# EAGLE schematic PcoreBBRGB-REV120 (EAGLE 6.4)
Assembly variants: FERT1S, FERT1B

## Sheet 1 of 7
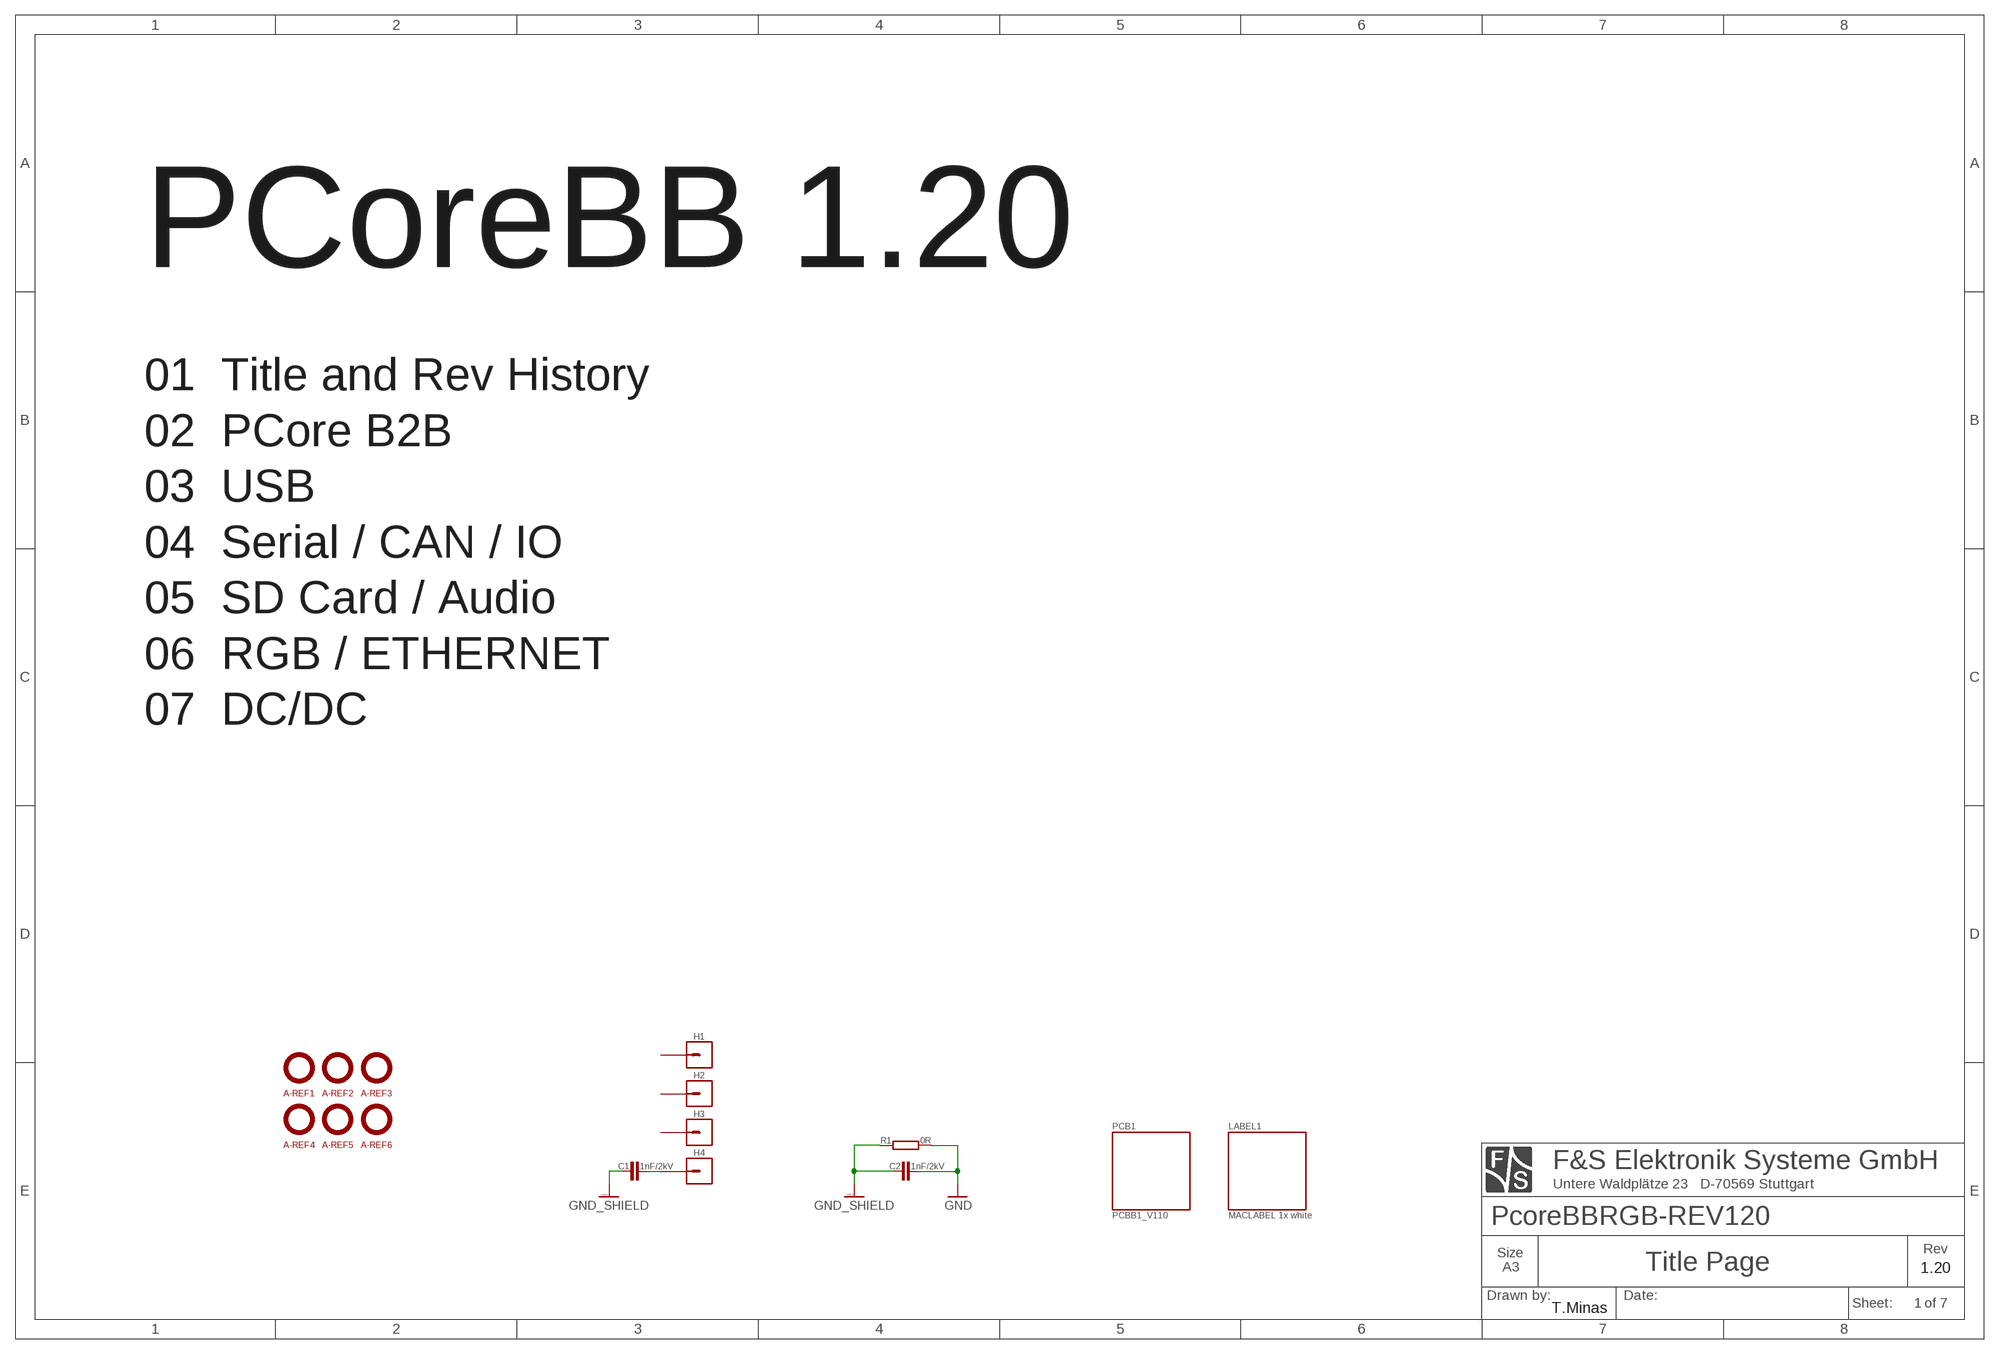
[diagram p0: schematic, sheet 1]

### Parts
A-REF1  A-REF  [A-REF]
A-REF2  A-REF  [A-REF]
A-REF3  A-REF  [A-REF]
A-REF4  A-REF  [A-REF]
A-REF5  A-REF  [A-REF]
A-REF6  A-REF  [A-REF]
C1  1nF/2kV  C1206-H  [1206]  (not fitted in variant FERT1B)
C2  1nF/2kV  C1206-H  [1206]  (not fitted in variant FERT1B)
H1  HOLE-3.2X6  [HOLE-3.2X6]  (not fitted in variant FERT1B)
H2  HOLE-3.2X6  [HOLE-3.2X6]  (not fitted in variant FERT1B)
H3  HOLE-3.2X6  [HOLE-3.2X6]  (not fitted in variant FERT1B)
H4  HOLE-3.2X6  [HOLE-3.2X6]  (not fitted in variant FERT1B)
R1  0R  R0805-H  [0805]  (not fitted in variant FERT1B)

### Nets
GND: C2.2 R1.2 ; also sheet 2,3,4,5,6,7
GND_SHIELD: C1.1 C2.1 R1.1 ; also sheet 3,6
N$1: C1.2 H4.P$1
Unconnected: H1.P$1 H2.P$1 H3.P$1

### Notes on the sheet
- PCoreBB 1.20
- 01  Title and Rev History
  02  PCore B2B
  03  USB
  04  Serial / CAN / IO
  05  SD Card / Audio
  06  RGB / ETHERNET
  07  DC/DC
- 1.20
- T.Minas

## Sheet 2 of 7: PicoCORE
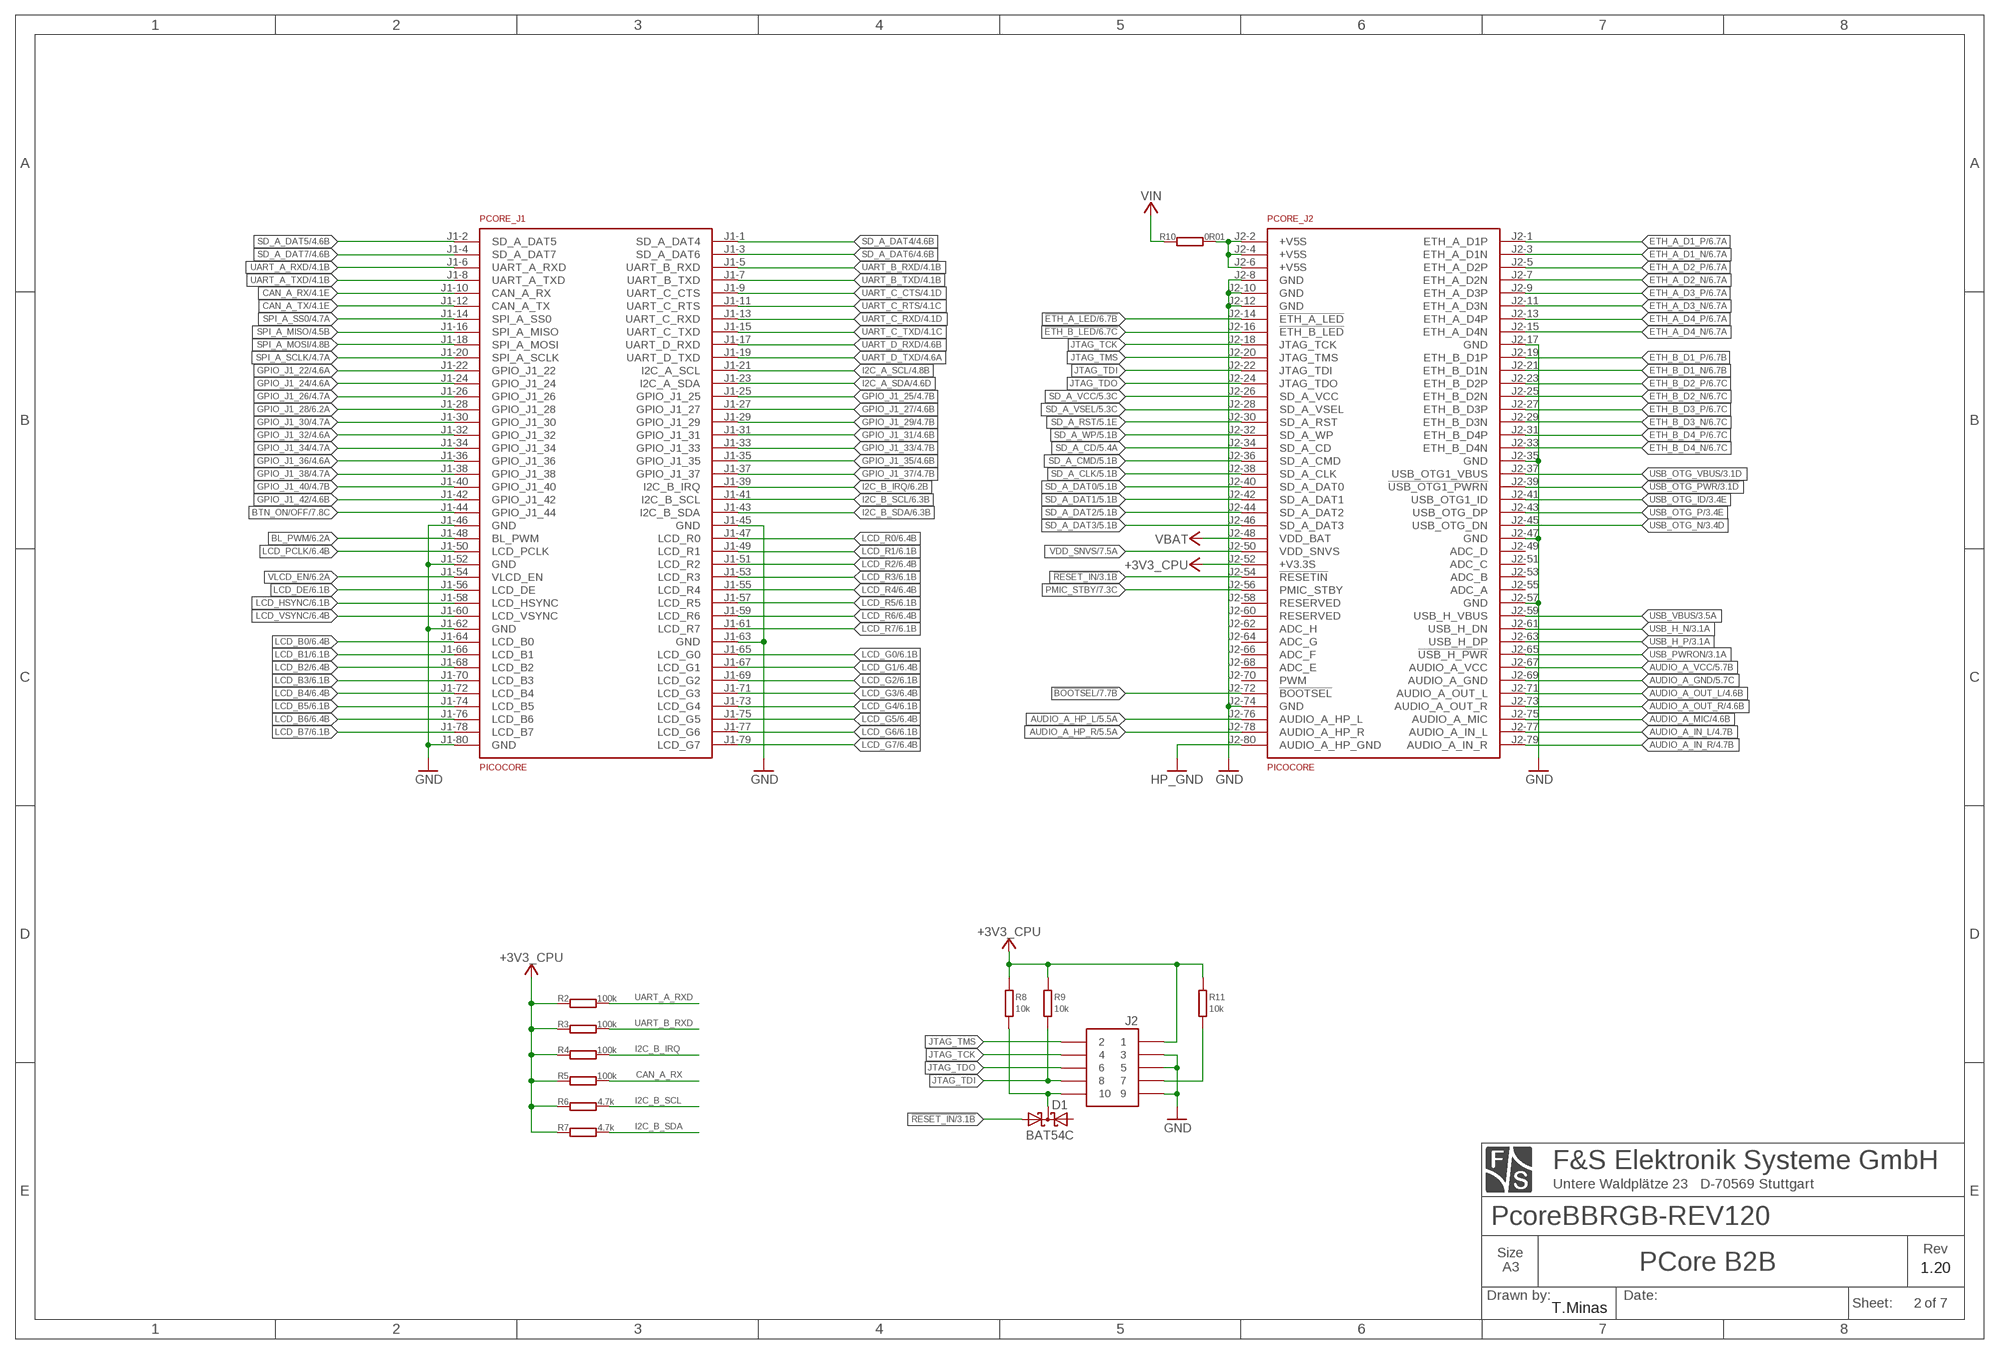
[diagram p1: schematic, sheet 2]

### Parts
D1  BAT54C  [SOT23]  (not fitted in variant FERT1B)
J2  CON-10-POL.-SMD-127  [10-POL.SMD-127]  (not fitted in variant FERT1B)
PCORE_  PICOCORE  [PICOCORE]  (not fitted in variant FERT1B)
R2  100k  R0402  [0402]  (not fitted in variant FERT1B)
R3  100k  R0402  [0402]  (not fitted in variant FERT1B)
R4  100k  R0402  [0402]  (not fitted in variant FERT1B)
R5  100k  R0402  [0402]  (not fitted in variant FERT1B)
R6  4.7k  R0402  [0402]  (not fitted in variant FERT1B)
R7  4.7k  R0402  [0402]  (not fitted in variant FERT1B)
R8  10k  R0402-V  [0402@1]  (not fitted in variant FERT1B)
R9  10k  R0402-V  [0402@1]  (not fitted in variant FERT1B)
R10  0R01  R0805-H  [0805]  (not fitted in variant FERT1B)
R11  10k  R0402-V  [0402@1]  (not fitted in variant FERT1B)

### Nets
!BOOTSEL: PCORE_.J2-72(J2:!BOOTSEL) ; also sheet 7
!ETH_A_LED: PCORE_.J2-14(J2:!ETH_A_LED) ; also sheet 6
!ETH_B_LED: PCORE_.J2-16(J2:!ETH_B_LED) ; also sheet 6
!JTAG_SRST: D1.3(CC) J2.10 R8.1
!RESET_IN: D1.1(A1) PCORE_.J2-54(J2:!RESETIN) ; also sheet 3,7
!USB_OTG_PWR: PCORE_.J2-39(J2:!USB_OTG1_PWRN) ; also sheet 3
+3V3_CPU [+3V3]: J2.1 PCORE_.J2-52(J2:+V3.3S) R2.1 R3.1 R4.1 R5.1 R6.1 R7.1 R8.2 R9.2 R11.2 ; also sheet 3,6,7
AUDIO_A_GND: PCORE_.J2-69(J2:AUDIO_A_GND) ; also sheet 5
AUDIO_A_HP_L: PCORE_.J2-76(J2:AUDIO_A_HP_L) ; also sheet 5
AUDIO_A_HP_R: PCORE_.J2-78(J2:AUDIO_A_HP_R) ; also sheet 5
AUDIO_A_IN_L: PCORE_.J2-77(J2:AUDIO_A_IN_L) ; also sheet 4
AUDIO_A_IN_R: PCORE_.J2-79(J2:AUDIO_A_IN_R) ; also sheet 4
AUDIO_A_MIC: PCORE_.J2-75(J2:AUDIO_A_MIC) ; also sheet 4,5
AUDIO_A_OUT_L: PCORE_.J2-71(J2:AUDIO_A_OUT_L) ; also sheet 4
AUDIO_A_OUT_R: PCORE_.J2-73(J2:AUDIO_A_OUT_R) ; also sheet 4
AUDIO_A_VCC: PCORE_.J2-67(J2:AUDIO_A_VCC) ; also sheet 5
BL_PWM: PCORE_.J1-48(J1:BL_PWM) ; also sheet 6
BTN_ON/OFF: PCORE_.J1-44(J1:GPIO_J1_44) ; also sheet 7
CAN_A_RX: PCORE_.J1-10(J1:CAN_A_RX) R5.2 ; also sheet 4
CAN_A_TX: PCORE_.J1-12(J1:CAN_A_TX) ; also sheet 4
ETH_A_D1_N [ETHERNET]: PCORE_.J2-3(J2:ETH_A_D1N) ; also sheet 6
ETH_A_D1_P [ETHERNET]: PCORE_.J2-1(J2:ETH_A_D1P) ; also sheet 6
ETH_A_D2_N [ETHERNET]: PCORE_.J2-7(J2:ETH_A_D2N) ; also sheet 6
ETH_A_D2_P [ETHERNET]: PCORE_.J2-5(J2:ETH_A_D2P) ; also sheet 6
ETH_A_D3_N [ETHERNET]: PCORE_.J2-11(J2:ETH_A_D3N) ; also sheet 6
ETH_A_D3_P [ETHERNET]: PCORE_.J2-9(J2:ETH_A_D3P) ; also sheet 6
ETH_A_D4_N [ETHERNET]: PCORE_.J2-15(J2:ETH_A_D4N) ; also sheet 6
ETH_A_D4_P [ETHERNET]: PCORE_.J2-13(J2:ETH_A_D4P) ; also sheet 6
ETH_B_D1_N [ETHERNET]: PCORE_.J2-21(J2:ETH_B_D1N) ; also sheet 6
ETH_B_D1_P [ETHERNET]: PCORE_.J2-19(J2:ETH_B_D1P) ; also sheet 6
ETH_B_D2_N [ETHERNET]: PCORE_.J2-25(J2:ETH_B_D2N) ; also sheet 6
ETH_B_D2_P [ETHERNET]: PCORE_.J2-23(J2:ETH_B_D2P) ; also sheet 6
ETH_B_D3_N [ETHERNET]: PCORE_.J2-29(J2:ETH_B_D3N) ; also sheet 6
ETH_B_D3_P [ETHERNET]: PCORE_.J2-27(J2:ETH_B_D3P) ; also sheet 6
ETH_B_D4_N [ETHERNET]: PCORE_.J2-33(J2:ETH_B_D4N) ; also sheet 6
ETH_B_D4_P [ETHERNET]: PCORE_.J2-31(J2:ETH_B_D4P) ; also sheet 6
GND: J2.3 J2.5 J2.9 PCORE_.J1-45(J1:GND) PCORE_.J1-46(J1:GND) PCORE_.J1-52(J1:GND) PCORE_.J1-62(J1:GND) PCORE_.J1-63(J1:GND) PCORE_.J1-80(J1:GND) PCORE_.J2-8(J2:GND) PCORE_.J2-10(J2:GND) PCORE_.J2-12(J2:GND) PCORE_.J2-17(J2:GND) PCORE_.J2-35(J2:GND) PCORE_.J2-47(J2:GND) PCORE_.J2-57(J2:GND) PCORE_.J2-74(J2:GND) ; also sheet 1,3,4,5,6,7
GPIO_J1_22: PCORE_.J1-22(J1:GPIO_J1_22) ; also sheet 4
GPIO_J1_24: PCORE_.J1-24(J1:GPIO_J1_24) ; also sheet 4
GPIO_J1_25: PCORE_.J1-25(J1:GPIO_J1_25) ; also sheet 4
GPIO_J1_26: PCORE_.J1-26(J1:GPIO_J1_26) ; also sheet 4
GPIO_J1_27: PCORE_.J1-27(J1:GPIO_J1_27) ; also sheet 4
GPIO_J1_28: PCORE_.J1-28(J1:GPIO_J1_28) ; also sheet 6
GPIO_J1_29: PCORE_.J1-29(J1:GPIO_J1_29) ; also sheet 4
GPIO_J1_30: PCORE_.J1-30(J1:GPIO_J1_30) ; also sheet 4
GPIO_J1_31: PCORE_.J1-31(J1:GPIO_J1_31) ; also sheet 4
GPIO_J1_32: PCORE_.J1-32(J1:GPIO_J1_32) ; also sheet 4
GPIO_J1_33: PCORE_.J1-33(J1:GPIO_J1_33) ; also sheet 4
GPIO_J1_34: PCORE_.J1-34(J1:GPIO_J1_34) ; also sheet 4
GPIO_J1_35: PCORE_.J1-35(J1:GPIO_J1_35) ; also sheet 4
GPIO_J1_36: PCORE_.J1-36(J1:GPIO_J1_36) ; also sheet 4
GPIO_J1_37: PCORE_.J1-37(J1:GPIO_J1_37) ; also sheet 4
GPIO_J1_38: PCORE_.J1-38(J1:GPIO_J1_38) ; also sheet 4
GPIO_J1_40: PCORE_.J1-40(J1:GPIO_J1_40) ; also sheet 4
GPIO_J1_42: PCORE_.J1-42(J1:GPIO_J1_42) ; also sheet 4
HP_GND: PCORE_.J2-80(J2:AUDIO_A_HP_GND) ; also sheet 5
I2C_A_SCL: PCORE_.J1-21(J1:I2C_A_SCL) ; also sheet 4
I2C_A_SDA: PCORE_.J1-23(J1:I2C_A_SDA) ; also sheet 4
I2C_B_IRQ: PCORE_.J1-39(J1:I2C_B_IRQ) R4.2 ; also sheet 6
I2C_B_SCL: PCORE_.J1-41(J1:I2C_B_SCL) R6.2 ; also sheet 6
I2C_B_SDA: PCORE_.J1-43(J1:I2C_B_SDA) R7.2 ; also sheet 6
JTAG_TCK: J2.4 PCORE_.J2-18(J2:JTAG_TCK)
JTAG_TDI: J2.8 PCORE_.J2-22(J2:JTAG_TDI) R9.1
JTAG_TDO: J2.6 PCORE_.J2-24(J2:JTAG_TDO)
JTAG_TMS: J2.2 PCORE_.J2-20(J2:JTAG_TMS)
LCD_B0: PCORE_.J1-64(J1:LCD_B0) ; also sheet 6
LCD_B1: PCORE_.J1-66(J1:LCD_B1) ; also sheet 6
LCD_B2: PCORE_.J1-68(J1:LCD_B2) ; also sheet 6
LCD_B3: PCORE_.J1-70(J1:LCD_B3) ; also sheet 6
LCD_B4: PCORE_.J1-72(J1:LCD_B4) ; also sheet 6
LCD_B5: PCORE_.J1-74(J1:LCD_B5) ; also sheet 6
LCD_B6: PCORE_.J1-76(J1:LCD_B6) ; also sheet 6
LCD_B7: PCORE_.J1-78(J1:LCD_B7) ; also sheet 6
LCD_DE: PCORE_.J1-56(J1:LCD_DE) ; also sheet 6
LCD_G0: PCORE_.J1-65(J1:LCD_G0) ; also sheet 6
LCD_G1: PCORE_.J1-67(J1:LCD_G1) ; also sheet 6
LCD_G2: PCORE_.J1-69(J1:LCD_G2) ; also sheet 6
LCD_G3: PCORE_.J1-71(J1:LCD_G3) ; also sheet 6
LCD_G4: PCORE_.J1-73(J1:LCD_G4) ; also sheet 6
LCD_G5: PCORE_.J1-75(J1:LCD_G5) ; also sheet 6
LCD_G6: PCORE_.J1-77(J1:LCD_G6) ; also sheet 6
LCD_G7: PCORE_.J1-79(J1:LCD_G7) ; also sheet 6
LCD_HSYNC: PCORE_.J1-58(J1:LCD_HSYNC) ; also sheet 6
LCD_PCLK: PCORE_.J1-50(J1:LCD_PCLK) ; also sheet 6
LCD_R0: PCORE_.J1-47(J1:LCD_R0) ; also sheet 6
LCD_R1: PCORE_.J1-49(J1:LCD_R1) ; also sheet 6
LCD_R2: PCORE_.J1-51(J1:LCD_R2) ; also sheet 6
LCD_R3: PCORE_.J1-53(J1:LCD_R3) ; also sheet 6
LCD_R4: PCORE_.J1-55(J1:LCD_R4) ; also sheet 6
LCD_R5: PCORE_.J1-57(J1:LCD_R5) ; also sheet 6
LCD_R6: PCORE_.J1-59(J1:LCD_R6) ; also sheet 6
LCD_R7: PCORE_.J1-61(J1:LCD_R7) ; also sheet 6
LCD_VSYNC: PCORE_.J1-60(J1:LCD_VSYNC) ; also sheet 6
N$23: PCORE_.J2-2(J2:+V5S) PCORE_.J2-4(J2:+V5S) PCORE_.J2-6(J2:+V5S) R10.2
N$34: J2.7 R11.1
PMIC_STBY: PCORE_.J2-56(J2:PMIC_STBY) ; also sheet 7
SD_A_CD: PCORE_.J2-34(J2:SD_A_CD) ; also sheet 5
SD_A_CLK: PCORE_.J2-38(J2:SD_A_CLK) ; also sheet 5
SD_A_CMD: PCORE_.J2-36(J2:SD_A_CMD) ; also sheet 5
SD_A_DAT0: PCORE_.J2-40(J2:SD_A_DAT0) ; also sheet 5
SD_A_DAT1: PCORE_.J2-42(J2:SD_A_DAT1) ; also sheet 5
SD_A_DAT2: PCORE_.J2-44(J2:SD_A_DAT2) ; also sheet 5
SD_A_DAT3: PCORE_.J2-46(J2:SD_A_DAT3) ; also sheet 5
SD_A_DAT4: PCORE_.J1-1(J1:SD_A_DAT4) ; also sheet 4
SD_A_DAT5: PCORE_.J1-2(J1:SD_A_DAT5) ; also sheet 4
SD_A_DAT6: PCORE_.J1-3(J1:SD_A_DAT6) ; also sheet 4
SD_A_DAT7: PCORE_.J1-4(J1:SD_A_DAT7) ; also sheet 4
SD_A_RST: PCORE_.J2-30(J2:SD_A_RST) ; also sheet 5
SD_A_VCC: PCORE_.J2-26(J2:SD_A_VCC) ; also sheet 5
SD_A_VSEL: PCORE_.J2-28(J2:SD_A_VSEL) ; also sheet 5
SD_A_WP: PCORE_.J2-32(J2:SD_A_WP) ; also sheet 5
SPI_A_MISO: PCORE_.J1-16(J1:SPI_A_MISO) ; also sheet 4
SPI_A_MOSI: PCORE_.J1-18(J1:SPI_A_MOSI) ; also sheet 4
SPI_A_SCLK: PCORE_.J1-20(J1:SPI_A_SCLK) ; also sheet 4
SPI_A_SS0: PCORE_.J1-14(J1:SPI_A_SS0) ; also sheet 4
UART_A_RXD: PCORE_.J1-6(J1:UART_A_RXD) R2.2 ; also sheet 4
UART_A_TXD: PCORE_.J1-8(J1:UART_A_TXD) ; also sheet 4
UART_B_RXD: PCORE_.J1-5(J1:UART_B_RXD) R3.2 ; also sheet 4
UART_B_TXD: PCORE_.J1-7(J1:UART_B_TXD) ; also sheet 4
UART_C_CTS: PCORE_.J1-9(J1:UART_C_CTS) ; also sheet 4
UART_C_RTS: PCORE_.J1-11(J1:UART_C_RTS) ; also sheet 4
UART_C_RXD: PCORE_.J1-13(J1:UART_C_RXD) ; also sheet 4
UART_C_TXD: PCORE_.J1-15(J1:UART_C_TXD) ; also sheet 4
UART_D_RXD: PCORE_.J1-17(J1:UART_D_RXD) ; also sheet 4
UART_D_TXD: PCORE_.J1-19(J1:UART_D_TXD) ; also sheet 4
USB_H_N [USB]: PCORE_.J2-61(J2:USB_H_DN) ; also sheet 3
USB_H_P [USB]: PCORE_.J2-63(J2:USB_H_DP) ; also sheet 3
USB_OTG_ID: PCORE_.J2-41(J2:USB_OTG1_ID) ; also sheet 3
USB_OTG_N [USB]: PCORE_.J2-45(J2:USB_OTG_DN) ; also sheet 3
USB_OTG_P [USB]: PCORE_.J2-43(J2:USB_OTG_DP) ; also sheet 3
USB_OTG_VBUS: PCORE_.J2-37(J2:USB_OTG1_VBUS) ; also sheet 3
USB_PWRON: PCORE_.J2-65(J2:!USB_H_PWR) ; also sheet 3
USB_VBUS: PCORE_.J2-59(J2:USB_H_VBUS) ; also sheet 3
VBAT: PCORE_.J2-48(J2:VDD_BAT) ; also sheet 7
VDD_SNVS: PCORE_.J2-50(J2:VDD_SNVS) ; also sheet 7
VIN: R10.1 ; also sheet 5,7
VLCD_EN: PCORE_.J1-54(J1:VLCD_EN) ; also sheet 6
Unconnected: D1.2(A2) PCORE_.J2-49(J2:ADC_D) PCORE_.J2-51(J2:ADC_C) PCORE_.J2-53(J2:ADC_B) PCORE_.J2-55(J2:ADC_A) PCORE_.J2-58(J2:RESERVED) PCORE_.J2-60(J2:RESERVED) PCORE_.J2-62(J2:ADC_H) PCORE_.J2-64(J2:ADC_G) PCORE_.J2-66(J2:ADC_F) PCORE_.J2-68(J2:ADC_E) PCORE_.J2-70(J2:PWM)

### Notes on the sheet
- 1.20
- T.Minas

## Sheet 3 of 7: USB
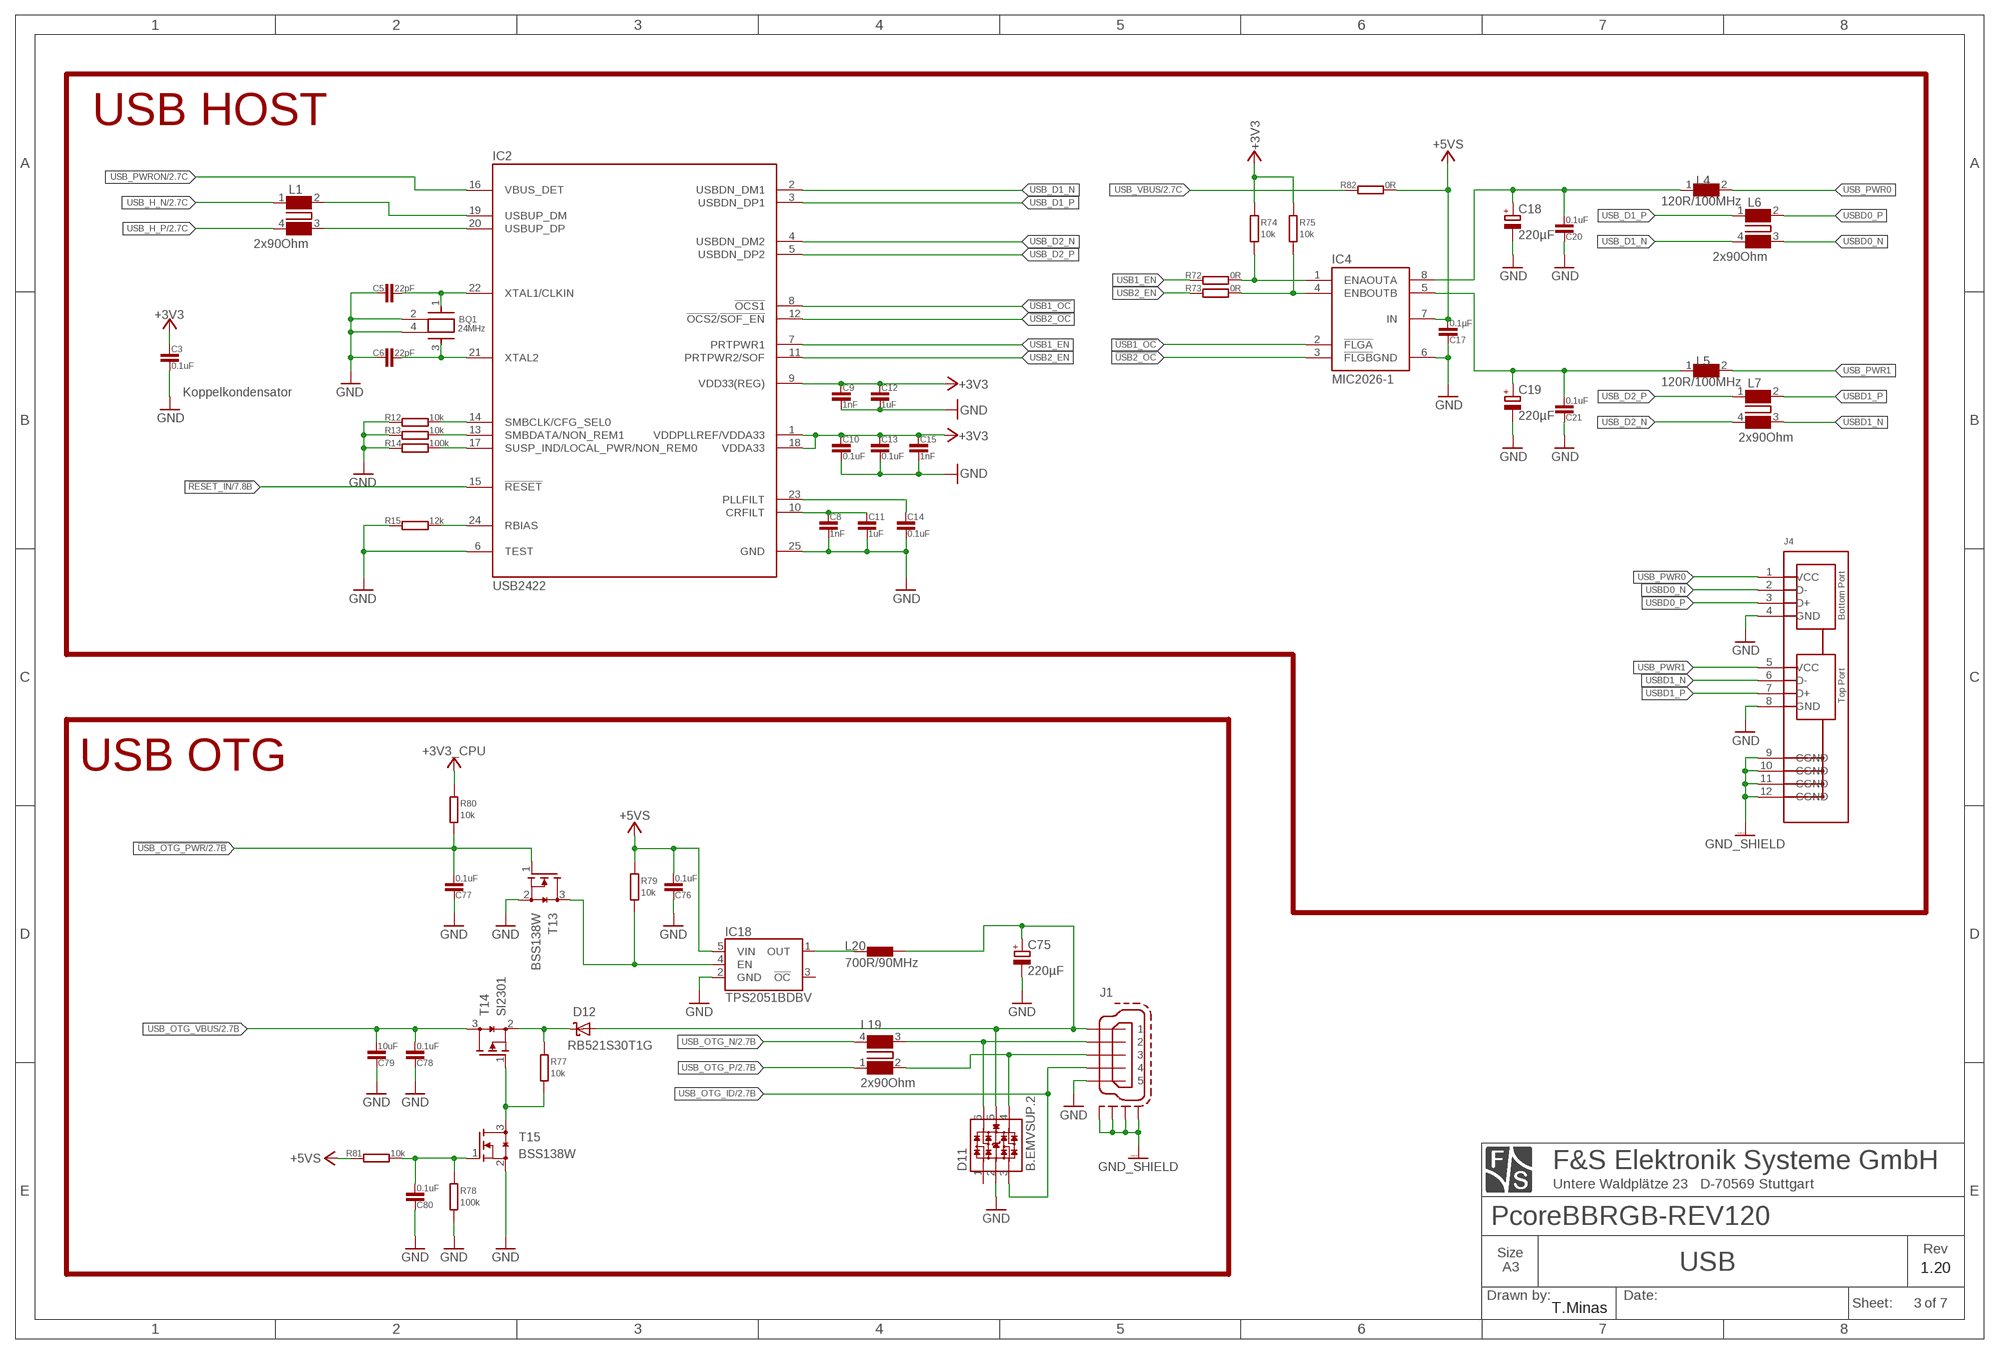
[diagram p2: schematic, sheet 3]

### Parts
BQ1  24MHz  Q-FA-238  [FA-238]  (not fitted in variant FERT1B)
C3  0.1uF  C0402-V  [0402@1]  (not fitted in variant FERT1B)
C5  22pF  C0402  [0402@1]  (not fitted in variant FERT1B)
C6  22pF  C0402  [0402@1]  (not fitted in variant FERT1B)
C8  1nF  C0402-V  [0402@1]  (not fitted in variant FERT1B)
C9  1nF  C0402-V  [0402@1]  (not fitted in variant FERT1B)
C10  0.1uF  C0402-V  [0402@1]  (not fitted in variant FERT1B)
C11  1uF  C0402-V  [0402@1]  (not fitted in variant FERT1B)
C12  1uF  C0402-V  [0402@1]  (not fitted in variant FERT1B)
C13  0.1uF  C0402-V  [0402@1]  (not fitted in variant FERT1B)
C14  0.1uF  C0402-V  [0402@1]  (not fitted in variant FERT1B)
C15  1nF  C0402-V  [0402@1]  (not fitted in variant FERT1B)
C17  0.1µF  C0402-V  [0402@1]  (not fitted in variant FERT1B)
C18  220µF  CPOL-EUSMCD  [SMC_D]  (not fitted in variant FERT1B)
C19  220µF  CPOL-EUSMCD  [SMC_D]  (not fitted in variant FERT1B)
C20  0.1uF  C0402-V  [0402@1]  (not fitted in variant FERT1B)
C21  0.1uF  C0402-V  [0402@1]  (not fitted in variant FERT1B)
C75  220µF  CPOL-EUSMCD  [SMC_D]  (not fitted in variant FERT1B)
C76  0.1uF  C0402-V  [0402@1]  (not fitted in variant FERT1B)
C77  0.1uF  C0402-V  [0402@1]  (not fitted in variant FERT1B)
C78  0.1uF  C0402-V  [0402@1]
C79  10uF  C0402-V  [0402@1]
C80  0.1uF  C0402-V  [0402@1]
D11  B.EMVSUP.2  ESD-PROTECTION-DIODE(4CHANNEL)  [SOT26]  (not fitted in variant FERT1B)
D12  RB521S30T1G  RB521S30  [SOD-523]
IC2  USB2422  [SQFN-24]  (not fitted in variant FERT1B)
IC4  MIC2026-1  MIC2026  [SO-8$1]  (not fitted in variant FERT1B)
IC18  TPS2051BDBV  [SOT23-5@1]  (not fitted in variant FERT1B)
J1  CON-MINI-USB-SCHIELD32005-201  [32005-201]  (not fitted in variant FERT1B)
J4  CON-USB-DOUBLE  [LUMBERG-2410-03]  (not fitted in variant FERT1S)
L1  2x90Ohm  WE-CNSW_HF_0805  [WE-CNSW_0805]  (not fitted in variant FERT1B)
L4  120R/100MHz  WE-CBF_HF_0402  [0402]  (not fitted in variant FERT1B)
L5  120R/100MHz  WE-CBF_HF_0402  [0402]  (not fitted in variant FERT1B)
L6  2x90Ohm  WE-CNSW_HF_0805  [WE-CNSW_0805]  (not fitted in variant FERT1B)
L7  2x90Ohm  WE-CNSW_HF_0805  [WE-CNSW_0805]  (not fitted in variant FERT1B)
L19  2x90Ohm  WE-CNSW_0805  [WE-CNSW_0805]  (not fitted in variant FERT1B)
L20  700R/90MHz  L-EU-1206  [1206]  (not fitted in variant FERT1B)
R12  10k  R0402  [0402]  (not fitted in variant FERT1B)
R13  10k  R0402  [0402]  (not fitted in variant FERT1B)
R14  100k  R0402  [0402]  (not fitted in variant FERT1B)
R15  12k  R0402  [0402]  (not fitted in variant FERT1B)
R72  0R  R0402  [0402]  (not fitted in variant FERT1B)
R73  0R  R0402  [0402]  (not fitted in variant FERT1B)
R74  10k  R0402-V  [0402@1]  (not fitted in variant FERT1B)  (not fitted in variant FERT1S)
R75  10k  R0402-V  [0402@1]  (not fitted in variant FERT1B)  (not fitted in variant FERT1S)
R77  10k  R0402-V  [0402@1]
R78  100k  R0402-V  [0402@1]
R79  10k  R0402-V  [0402@1]  (not fitted in variant FERT1B)
R80  10k  R0402-V  [0402@1]  (not fitted in variant FERT1B)
R81  10k  R0402  [0402]
R82  0R  R0402  [0402]
T13  BSS138W  [SOT323(SC70)]  (not fitted in variant FERT1B)
T14  SI2301  SI2301DS  [SOT23]
T15  BSS138W  [SOT323(SC70)]

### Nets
!RESET_IN: IC2.15(!RESET) ; also sheet 2,7
!USB1_OC: IC2.8(!OCS1) IC4.2(!FLGA)
!USB2_OC: IC2.12(!OCS2!/!SOF_EN) IC4.3(!FLGB)
!USB_OTG_PWR: C77.2 R80.1 T13.1(G) ; also sheet 2
+3V3 [+3V3]: C3.1 C9.1 C10.1 C12.1 C13.1 C15.1 IC2.1(VDDPLLREF/VDDA33) IC2.9(VDD33(REG)) IC2.18(VDDA33) R74.2 R75.2 ; also sheet 4,5,6,7
+3V3_CPU [+3V3]: R80.2 ; also sheet 2,6,7
+5VS: C17.2 C76.2 IC4.7(IN) IC18.5(VIN) R79.2 R81.1 R82.2 ; also sheet 4,6,7
GND: BQ1.2 BQ1.4 C3.2 C5.1 C6.1 C8.2 C9.2 C10.2 C11.2 C12.2 C13.2 C14.2 C15.2 C17.1 C18.- C19.- C20.1 C21.1 C75.- C76.1 C77.1 C78.1 C79.1 C80.1 D11.2 IC2.6(TEST) IC2.25(GND) IC4.6(GND) IC18.2(GND) J1.5 J4.4(GND) J4.8(GND) R12.1 R13.1 R14.1 R15.1 R78.1 T13.2(S) T15.2(S) ; also sheet 1,2,4,5,6,7
GND_SHIELD: J1.M1(S1) J1.M2(S2) J1.M3(S3) J1.M4(S4) J4.9(CGND) J4.10(CGND) J4.11(CGND) J4.12(CGND) ; also sheet 1,6
N$43: IC4.1(ENA) R72.2 R74.1
N$45: IC4.4(ENB) R73.2 R75.1
N$50: C75.+ D11.5 D12.2(A) J1.1 L20.1(IN)
N$51: IC18.1(OUT) L20.2(OUT)
N$52: D12.1(C) R77.2 T14.2(S)
N$54: IC18.4(EN) R79.1 T13.3(D)
N$55: R77.1 T14.1(G) T15.3(D)
N$56: C80.2 R78.2 R81.2 T15.1(G)
N$69: C18.+ C20.2 IC4.8(OUTA) L4.1
N$70: C19.+ C21.2 IC4.5(OUTB) L5.1
N$71: IC2.17(SUSP_IND/LOCAL_PWR/NON_REM0) R14.2
N$73: IC2.13(SMBDATA/NON_REM1) R13.2
N$74: BQ1.3 C6.2 IC2.21(XTAL2)
N$77: BQ1.1 C5.2 IC2.22(XTAL1/CLKIN)
N$86: IC2.14(SMBCLK/CFG_SEL0) R12.2
N$87: IC2.24(RBIAS) R15.2
N$88: C8.1 C11.1 IC2.10(CRFILT)
N$89: C14.1 IC2.23(PLLFILT)
USB1_EN: IC2.7(PRTPWR1) R72.1
USB1_N [USB]: IC2.19(USBUP_DM) L1.2
USB1_P [USB]: IC2.20(USBUP_DP) L1.3
USB2_EN: IC2.11(PRTPWR2/SOF) R73.1
USB-D1_N [USB]: D11.6 J1.2 L19.3
USB-D1_P [USB]: D11.4 J1.3 L19.2
USB_D1_N [USB]: IC2.2(USBDN_DM1) L6.4
USB_D1_P [USB]: IC2.3(USBDN_DP1) L6.1
USB_D2_N [USB]: IC2.4(USBDN_DM2) L7.4
USB_D2_P [USB]: IC2.5(USBDN_DP2) L7.1
USB_H_N [USB]: L1.1 ; also sheet 2
USB_H_P [USB]: L1.4 ; also sheet 2
USB_OTG_ID: D11.3 J1.4 ; also sheet 2
USB_OTG_N [USB]: L19.4 ; also sheet 2
USB_OTG_P [USB]: L19.1 ; also sheet 2
USB_OTG_VBUS: C78.2 C79.2 T14.3(D) ; also sheet 2
USB_PWR0: J4.1(VCC) L4.2
USB_PWR1: J4.5(VCC) L5.2
USB_PWRON: IC2.16(VBUS_DET) ; also sheet 2
USB_VBUS: R82.1 ; also sheet 2
USBD0_N [USB]: J4.2(D-) L6.3
USBD0_P [USB]: J4.3(D+) L6.2
USBD1_N [USB]: J4.6(D-) L7.3
USBD1_P [USB]: J4.7(D+) L7.2
Unconnected: D11.1 IC18.3(!OC)

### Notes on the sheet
- USB HOST
- Koppelkondensator
- USB OTG
- 1.20
- T.Minas

## Sheet 4 of 7: Serial / CAN / IO
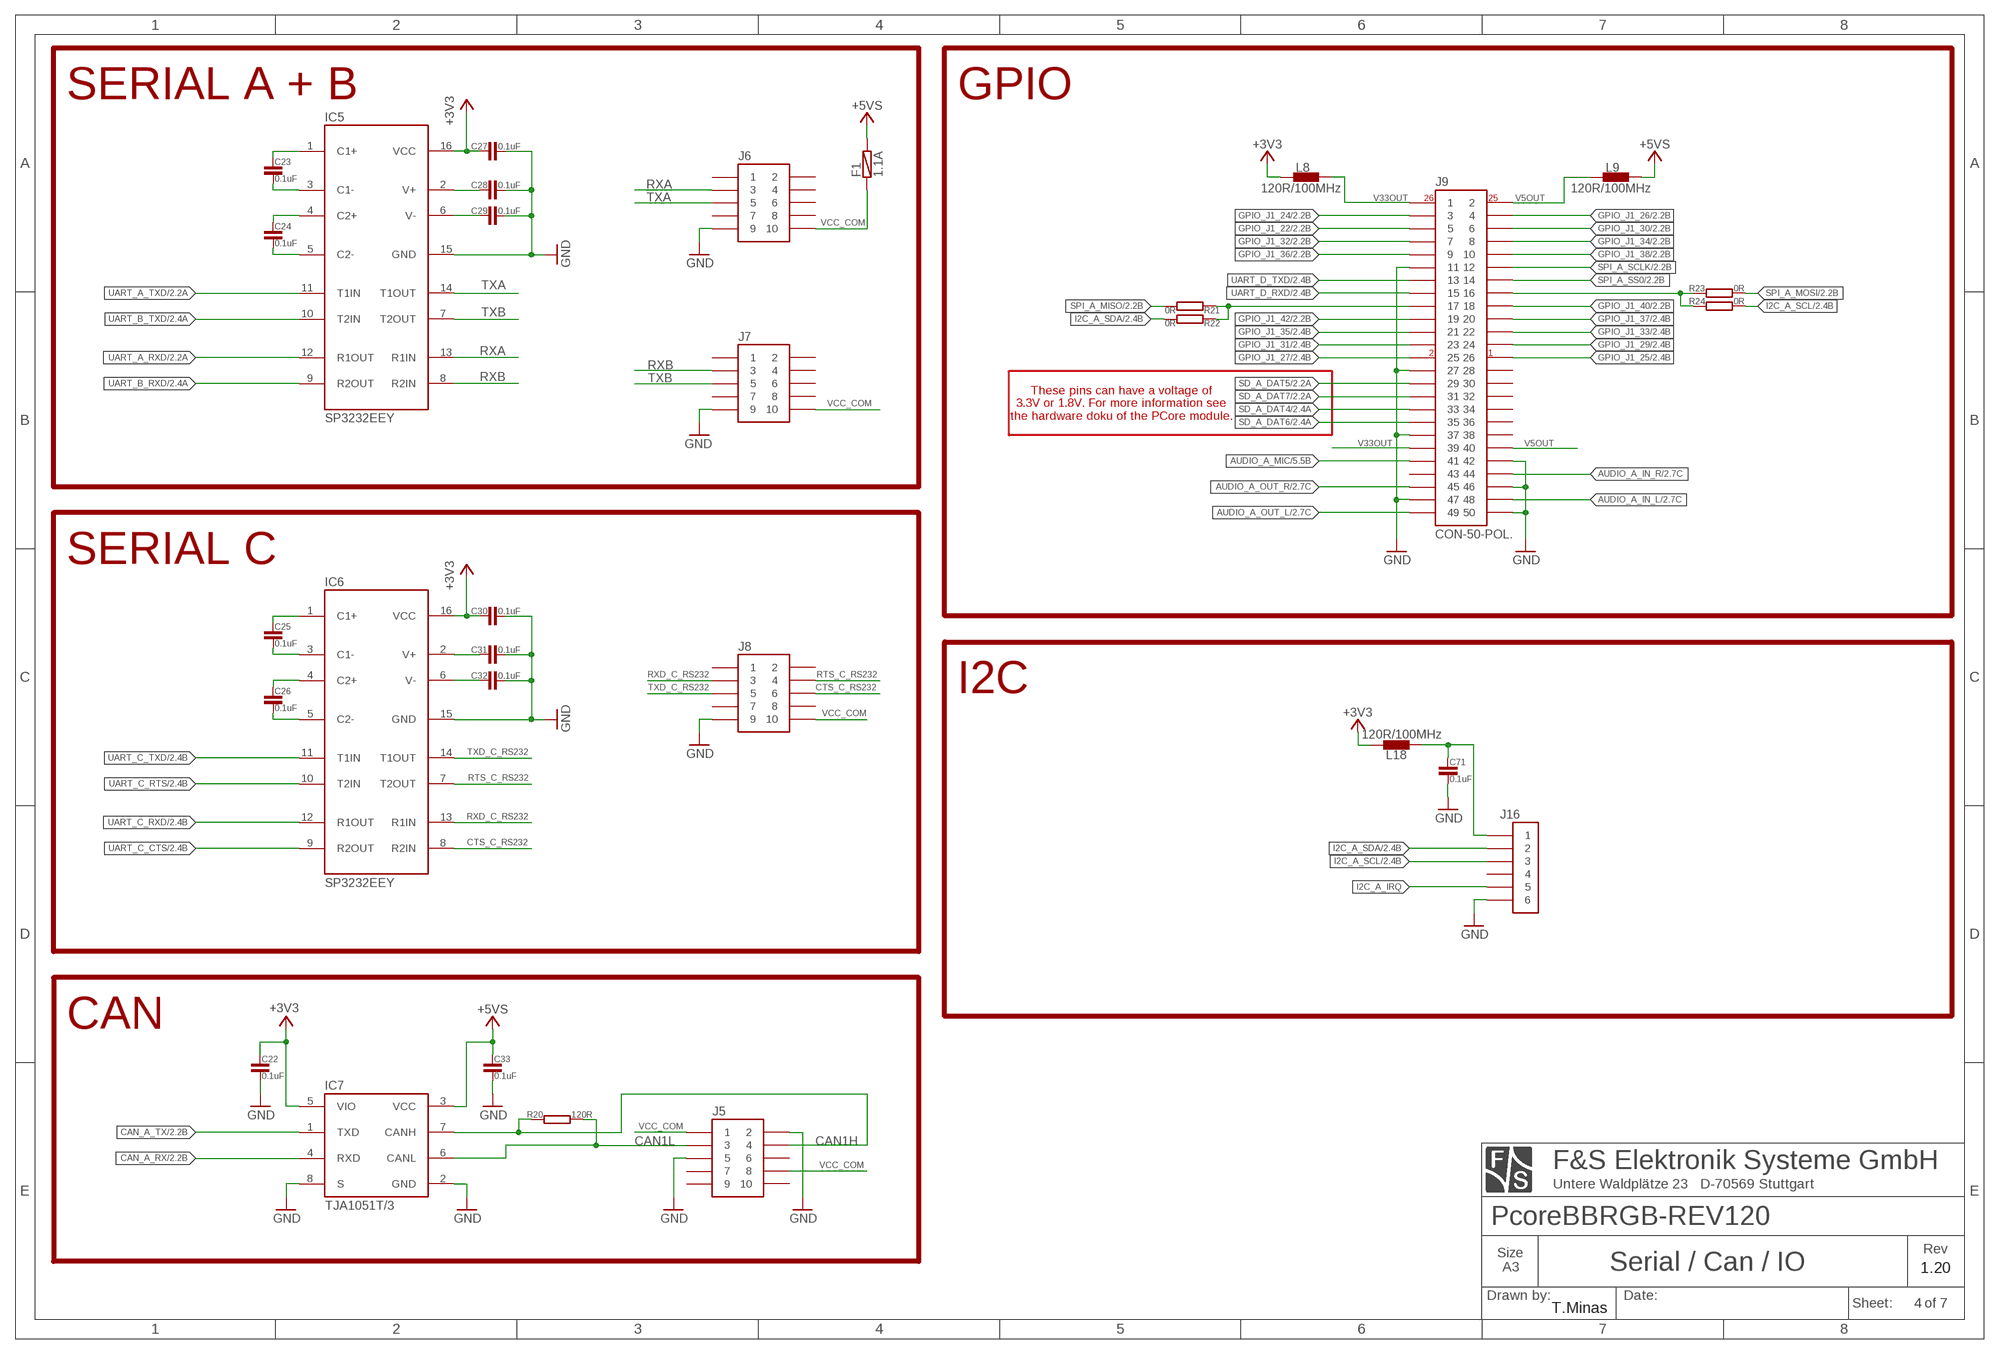
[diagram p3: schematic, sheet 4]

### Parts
C22  0.1uF  C0402-V  [0402@1]  (not fitted in variant FERT1B)
C23  0.1uF  C0402-V  [0402@1]  (not fitted in variant FERT1B)
C24  0.1uF  C0402-V  [0402@1]  (not fitted in variant FERT1B)
C25  0.1uF  C0402-V  [0402@1]  (not fitted in variant FERT1B)
C26  0.1uF  C0402-V  [0402@1]  (not fitted in variant FERT1B)
C27  0.1uF  C0402  [0402@1]  (not fitted in variant FERT1B)
C28  0.1uF  C0402  [0402@1]  (not fitted in variant FERT1B)
C29  0.1uF  C0402  [0402@1]  (not fitted in variant FERT1B)
C30  0.1uF  C0402  [0402@1]  (not fitted in variant FERT1B)
C31  0.1uF  C0402  [0402@1]  (not fitted in variant FERT1B)
C32  0.1uF  C0402  [0402@1]  (not fitted in variant FERT1B)
C33  0.1uF  C0402-V  [0402@1]  (not fitted in variant FERT1B)
C71  0.1uF  C0402-V  [0402@1]
F1  1.1A  F-EU-0805  [0805]  (not fitted in variant FERT1B)
IC5  SP3232EEY  SP3232ECY  [TSSOP-16]  (not fitted in variant FERT1B)
IC6  SP3232EEY  SP3232ECY  [TSSOP-16]  (not fitted in variant FERT1B)
IC7  TJA1051T/3  [SO-8]  (not fitted in variant FERT1B)
J5  CON-10-POL.-STIFTWANNE-B  [CON-10POL.-STIFTWANNE]  (not fitted in variant FERT1S)
J6  CON-10-POL.-STIFTWANNE-B  [CON-10POL.-STIFTWANNE]  (not fitted in variant FERT1S)
J7  CON-10-POL.-STIFTWANNE-B  [CON-10POL.-STIFTWANNE]  (not fitted in variant FERT1S)
J8  CON-10-POL.-STIFTWANNE-B  [CON-10POL.-STIFTWANNE]  (not fitted in variant FERT1S)
J9  CON-50-POL.  [50-POL.]  (not fitted in variant FERT1S)
J16  CON-HIROSE-DF13A-6P  [CON-HIROSE-DF13A-6P]  (not fitted in variant FERT1B)
L8  120R/100MHz  L-EU-0603  [0603]  (not fitted in variant FERT1B)
L9  120R/100MHz  L-EU-0603  [0603]  (not fitted in variant FERT1B)
L18  120R/100MHz  L-EU-0603  [0603]  (not fitted in variant FERT1B)
R20  120R  R0402  [0402]  (not fitted in variant FERT1B)
R21  0R  R0402  [0402]  (not fitted in variant FERT1B)
R22  0R  R0402  [0402]  (not fitted in variant FERT1B)  (not fitted in variant FERT1S)
R23  0R  R0402  [0402]  (not fitted in variant FERT1B)
R24  0R  R0402  [0402]  (not fitted in variant FERT1B)  (not fitted in variant FERT1S)

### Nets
+3V3 [+3V3]: C22.1 C27.1 C30.1 IC5.16(VCC) IC6.16(VCC) IC7.5(VIO) L8.1(IN) L18.2(OUT) ; also sheet 3,5,6,7
+5VS: C33.1 F1.1(IN) IC7.3(VCC) L9.2(OUT) ; also sheet 3,6,7
AUDIO_A_IN_L: J9.48 ; also sheet 2
AUDIO_A_IN_R: J9.44 ; also sheet 2
AUDIO_A_MIC: J9.41 ; also sheet 2,5
AUDIO_A_OUT_L: J9.49 ; also sheet 2
AUDIO_A_OUT_R: J9.45 ; also sheet 2
CAN1H: IC7.7(CANH) J5.4 R20.1
CAN1L: IC7.6(CANL) J5.3 R20.2
CAN_A_RX: IC7.4(RXD) ; also sheet 2
CAN_A_TX: IC7.1(TXD) ; also sheet 2
CTS_C_RS232: IC6.8(R2IN) J8.6
GND: C22.2 C27.2 C28.2 C29.2 C30.2 C31.2 C32.2 C33.2 C71.2 IC5.15(GND) IC6.15(GND) IC7.2(GND) IC7.8(S) J5.2 J5.5 J6.9 J7.9 J8.9 J9.11 J9.27 J9.37 J9.42 J9.46 J9.47 J9.50 J16.6 ; also sheet 1,2,3,5,6,7
GPIO_J1_22: J9.5 ; also sheet 2
GPIO_J1_24: J9.3 ; also sheet 2
GPIO_J1_25: J9.26 ; also sheet 2
GPIO_J1_26: J9.4 ; also sheet 2
GPIO_J1_27: J9.25 ; also sheet 2
GPIO_J1_29: J9.24 ; also sheet 2
GPIO_J1_30: J9.6 ; also sheet 2
GPIO_J1_31: J9.23 ; also sheet 2
GPIO_J1_32: J9.7 ; also sheet 2
GPIO_J1_33: J9.22 ; also sheet 2
GPIO_J1_34: J9.8 ; also sheet 2
GPIO_J1_35: J9.21 ; also sheet 2
GPIO_J1_36: J9.9 ; also sheet 2
GPIO_J1_37: J9.20 ; also sheet 2
GPIO_J1_38: J9.10 ; also sheet 2
GPIO_J1_40: J9.18 ; also sheet 2
GPIO_J1_42: J9.19 ; also sheet 2
I2C_A_IRQ: J16.5
I2C_A_SCL: J16.3 R24.2 ; also sheet 2
I2C_A_SDA: J16.2 R22.2 ; also sheet 2
N$2: J9.17 R21.1 R22.1
N$4: J9.16 R23.1 R24.1
N$8: C23.1 IC5.1(C1+)
N$9: C23.2 IC5.3(C1-)
N$10: C24.2 IC5.5(C2-)
N$11: C24.1 IC5.4(C2+)
N$13: C28.1 IC5.2(V+)
N$14: C29.1 IC5.6(V-)
N$17: C25.1 IC6.1(C1+)
N$21: C25.2 IC6.3(C1-)
N$26: C71.1 J16.1 L18.1(IN)
N$28: C26.2 IC6.5(C2-)
N$30: C26.1 IC6.4(C2+)
N$31: C31.1 IC6.2(V+)
N$32: C32.1 IC6.6(V-)
RTS_C_RS232: IC6.7(T2OUT) J8.4
RXA: IC5.13(R1IN) J6.3
RXB: IC5.8(R2IN) J7.3
RXD_C_RS232: IC6.13(R1IN) J8.3
SD_A_DAT4: J9.33 ; also sheet 2
SD_A_DAT5: J9.29 ; also sheet 2
SD_A_DAT6: J9.35 ; also sheet 2
SD_A_DAT7: J9.31 ; also sheet 2
SPI_A_MISO: R21.2 ; also sheet 2
SPI_A_MOSI: R23.2 ; also sheet 2
SPI_A_SCLK: J9.12 ; also sheet 2
SPI_A_SS0: J9.14 ; also sheet 2
TXA: IC5.14(T1OUT) J6.5
TXB: IC5.7(T2OUT) J7.5
TXD_C_RS232: IC6.14(T1OUT) J8.5
UART_A_RXD: IC5.12(R1OUT) ; also sheet 2
UART_A_TXD: IC5.11(T1IN) ; also sheet 2
UART_B_RXD: IC5.9(R2OUT) ; also sheet 2
UART_B_TXD: IC5.10(T2IN) ; also sheet 2
UART_C_CTS: IC6.9(R2OUT) ; also sheet 2
UART_C_RTS: IC6.10(T2IN) ; also sheet 2
UART_C_RXD: IC6.12(R1OUT) ; also sheet 2
UART_C_TXD: IC6.11(T1IN) ; also sheet 2
UART_D_RXD: J9.15 ; also sheet 2
UART_D_TXD: J9.13 ; also sheet 2
V5OUT: J9.2 J9.40 L9.1(IN)
V33OUT: J9.1 J9.39 L8.2(OUT)
VCC_COM: F1.2(OUT) J5.1 J5.8 J6.10 J7.10 J8.10
Unconnected: J5.6 J5.7 J5.9 J5.10 J6.1 J6.2 J6.4 J6.6 J6.7 J6.8 J7.1 J7.2 J7.4 J7.6 J7.7 J7.8 J8.1 J8.2 J8.7 J8.8 J9.28 J9.30 J9.32 J9.34 J9.36 J9.38 J9.43 J16.4

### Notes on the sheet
- SERIAL A + B | GPIO
- 26
- 25
- 2
- 1
- These pins can have a voltage of
  3.3V or 1.8V. For more information see
  the hardware doku of the PCore module.
- SERIAL C
- I2C
- CAN
- 1.20
- T.Minas

## Sheet 5 of 7: SD Card / Audio
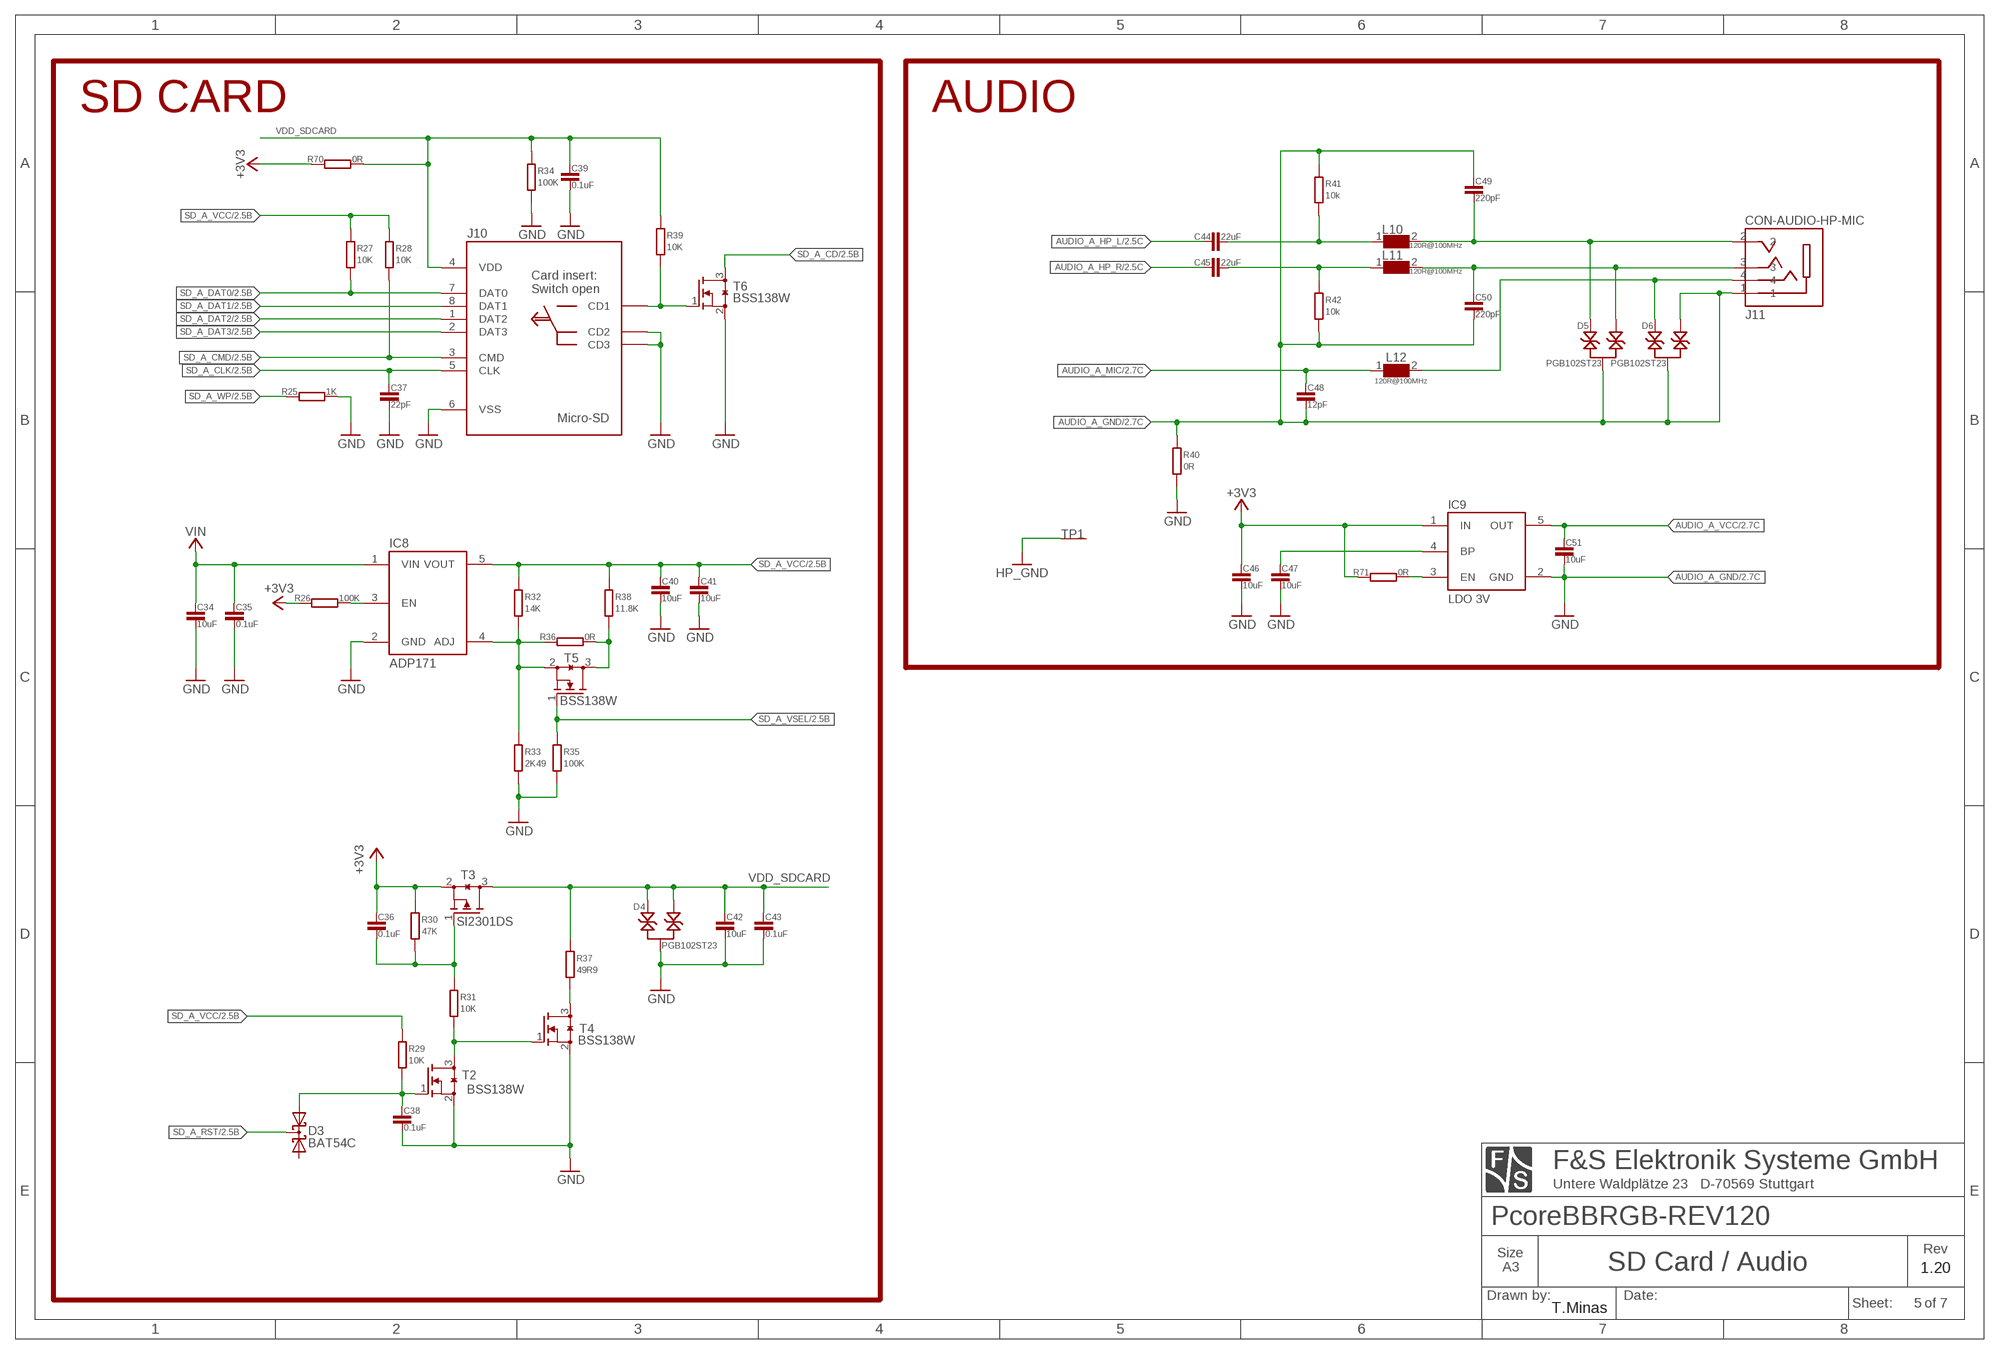
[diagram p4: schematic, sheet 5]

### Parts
C34  10uF  C0402-V  [0402@1]  (not fitted in variant FERT1B)
C35  0.1uF  C0402-V  [0402@1]  (not fitted in variant FERT1B)
C36  0.1uF  C0402-V  [0402@1]  (not fitted in variant FERT1B)
C37  22pF  C0402-V  [0402@1]  (not fitted in variant FERT1B)
C38  0.1uF  C0402-V  [0402@1]  (not fitted in variant FERT1B)
C39  0.1uF  C0402-V  [0402@1]  (not fitted in variant FERT1B)
C40  10uF  C0402-V  [0402@1]  (not fitted in variant FERT1B)
C41  10uF  C0402-V  [0402@1]  (not fitted in variant FERT1B)
C42  10uF  C0402-V  [0402@1]  (not fitted in variant FERT1B)
C43  0.1uF  C0402-V  [0402@1]  (not fitted in variant FERT1B)
C44  22uF  C0603-H  [0603]  (not fitted in variant FERT1B)
C45  22uF  C0603-H  [0603]  (not fitted in variant FERT1B)
C46  10uF  C0402-V  [0402@1]  (not fitted in variant FERT1B)
C47  10uF  C0402-V  [0402@1]  (not fitted in variant FERT1B)
C48  12pF  C0402-V  [0402@1]  (not fitted in variant FERT1B)
C49  220pF  C0402-V  [0402@1]  (not fitted in variant FERT1B)
C50  220pF  C0402-V  [0402@1]  (not fitted in variant FERT1B)
C51  10uF  C0402-V  [0402@1]  (not fitted in variant FERT1B)
D3  BAT54C  [SOT23]  (not fitted in variant FERT1B)
D4  PGB102ST23  PGB1SOT23  [SOT-23]  (not fitted in variant FERT1B)
D5  PGB102ST23  PGB1SOT23  [SOT-23]  (not fitted in variant FERT1B)
D6  PGB102ST23  PGB1SOT23  [SOT-23]  (not fitted in variant FERT1B)
IC8  ADP171  [SOT23-5]  (not fitted in variant FERT1B)
IC9  LDO 3V  AP7365  [SOT23-5]  (not fitted in variant FERT1B)
J10  CON-MICRO-SD-PUSHPULL  [MICRO-SD-PUSHPULL]  (not fitted in variant FERT1B)
J11  CON-AUDIO-HP-MIC  [CON-AUDIO-SJ2]  (not fitted in variant FERT1B)
L10  120R@100MHz  WE-CBF_HF_0402  [0402]  (not fitted in variant FERT1B)
L11  120R@100MHz  WE-CBF_HF_0402  [0402]  (not fitted in variant FERT1B)
L12  120R@100MHz  WE-CBF_HF_0402  [0402]  (not fitted in variant FERT1B)
R25  1K  R0402  [0402]  (not fitted in variant FERT1B)
R26  100K  R0402  [0402]  (not fitted in variant FERT1B)
R27  10K  R0402-V  [0402@1]  (not fitted in variant FERT1B)
R28  10K  R0402-V  [0402@1]  (not fitted in variant FERT1B)
R29  10K  R0402-V  [0402@1]  (not fitted in variant FERT1B)
R30  47K  R0402-V  [0402@1]  (not fitted in variant FERT1B)
R31  10K  R0402-V  [0402@1]  (not fitted in variant FERT1B)
R32  14K  R0402-V  [0402@1]  (not fitted in variant FERT1B)
R33  2K49  R0402-V  [0402@1]  (not fitted in variant FERT1B)
R34  100K  R0402-V  [0402@1]  (not fitted in variant FERT1B)
R35  100K  R0402-V  [0402@1]  (not fitted in variant FERT1B)
R36  0R  R0402  [0402]  (not fitted in variant FERT1B)  (not fitted in variant FERT1S)
R37  49R9  R0402-V  [0402@1]  (not fitted in variant FERT1B)
R38  11.8K  R0402-V  [0402@1]  (not fitted in variant FERT1B)
R39  10K  R0402-V  [0402@1]  (not fitted in variant FERT1B)
R40  0R  R0402-V  [0402@1]  (not fitted in variant FERT1B)
R41  10k  R0402-V  [0402@1]  (not fitted in variant FERT1B)
R42  10k  R0402-V  [0402@1]  (not fitted in variant FERT1B)
R70  0R  R0402  [0402]  (not fitted in variant FERT1S)  (not fitted in variant FERT1B)
R71  0R  R0402  [0402]  (not fitted in variant FERT1B)
T2  BSS138W  [SOT323(SC70)]  (not fitted in variant FERT1B)
T3  SI2301DS  [SOT23]  (not fitted in variant FERT1B)
T4  BSS138W  [SOT323(SC70)]  (not fitted in variant FERT1B)
T5  BSS138W  [SOT323(SC70)]  (not fitted in variant FERT1B)
T6  BSS138W  [SOT323(SC70)]  (not fitted in variant FERT1B)
TP1  TEST2  [TEST2]  (not fitted in variant FERT1B)

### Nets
+3V3 [+3V3]: C36.1 C46.1 IC9.1(IN) R26.1 R30.2 R70.1 R71.1 T3.2(S) ; also sheet 3,4,6,7
AUDIO_A_GND: C48.2 C49.1 C50.2 C51.2 D5.3 D6.1 D6.3 IC9.2(GND) J11.1 R40.2 R41.2 R42.1 ; supply symbol labelled GND ; also sheet 2
AUDIO_A_HP_L: C44.1 ; also sheet 2
AUDIO_A_HP_R: C45.1 ; also sheet 2
AUDIO_A_MIC: C48.1 L12.1 ; also sheet 2,4
AUDIO_A_VCC: C51.1 IC9.5(OUT) ; also sheet 2
GND: C34.2 C35.2 C37.2 C38.2 C39.2 C40.2 C41.2 C42.2 C43.2 C46.2 C47.2 D4.3 IC8.2(GND) J10.6(VSS) J10.10@1(CD2) J10.10@2(CD3) R25.2 R33.1 R34.1 R35.1 R40.1 T2.2(S) T4.2(S) T6.2(S) ; also sheet 1,2,3,4,6,7
HP_GND: TP1.P$1 ; also sheet 2
N$12: R31.1 T2.3(D) T4.1(G)
N$15: J10.9@1(CD1) J10.9@2(CD1) R39.1 T6.1(G)
N$16: C38.1 D3.2(A2) R29.1 T2.1(G)
N$18: R37.1 T4.3(D)
N$19: IC8.3(EN) R26.2
N$20: C36.2 R30.1 R31.2 T3.1(G)
N$24: IC8.4(ADJ) R32.1 R33.2 R36.1 T5.2(S)
N$25: R36.2 R38.1 T5.3(D)
N$27 [+3V3]: IC9.3(EN) R71.2
N$33: C45.2 L11.1 R42.2
N$35: C44.2 L10.1 R41.1
N$39: C49.2 D5.2 J11.2 L10.2
N$40: C50.1 D5.1 J11.3 L11.2
N$42: C47.1 IC9.4(BP)
N$46: D6.2 J11.4 L12.2
SD_A_CD: T6.3(D) ; also sheet 2
SD_A_CLK: C37.1 J10.5(CLK) ; also sheet 2
SD_A_CMD: J10.3(CMD) R28.1 ; also sheet 2
SD_A_DAT0: J10.7(DAT0) R27.1 ; also sheet 2
SD_A_DAT1: J10.8(DAT1) ; also sheet 2
SD_A_DAT2: J10.1(DAT2) ; also sheet 2
SD_A_DAT3: J10.2(DAT3) ; also sheet 2
SD_A_RST: D3.3(CC) ; also sheet 2
SD_A_VCC: C40.1 C41.1 IC8.5(VOUT) R27.2 R28.2 R29.2 R32.2 R38.2 ; also sheet 2
SD_A_VSEL: R35.2 T5.1(G) ; also sheet 2
SD_A_WP: R25.1 ; also sheet 2
VDD_SDCARD: C39.1 C42.1 C43.1 D4.1 D4.2 J10.4(VDD) R34.2 R37.2 R39.2 R70.2 T3.3(D)
VIN: C34.1 C35.1 IC8.1(VIN) ; also sheet 2,7
Unconnected: D3.1(A1)

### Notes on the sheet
- SD CARD | AUDIO
- 1.20
- T.Minas

## Sheet 6 of 7: RGB / Ethernet
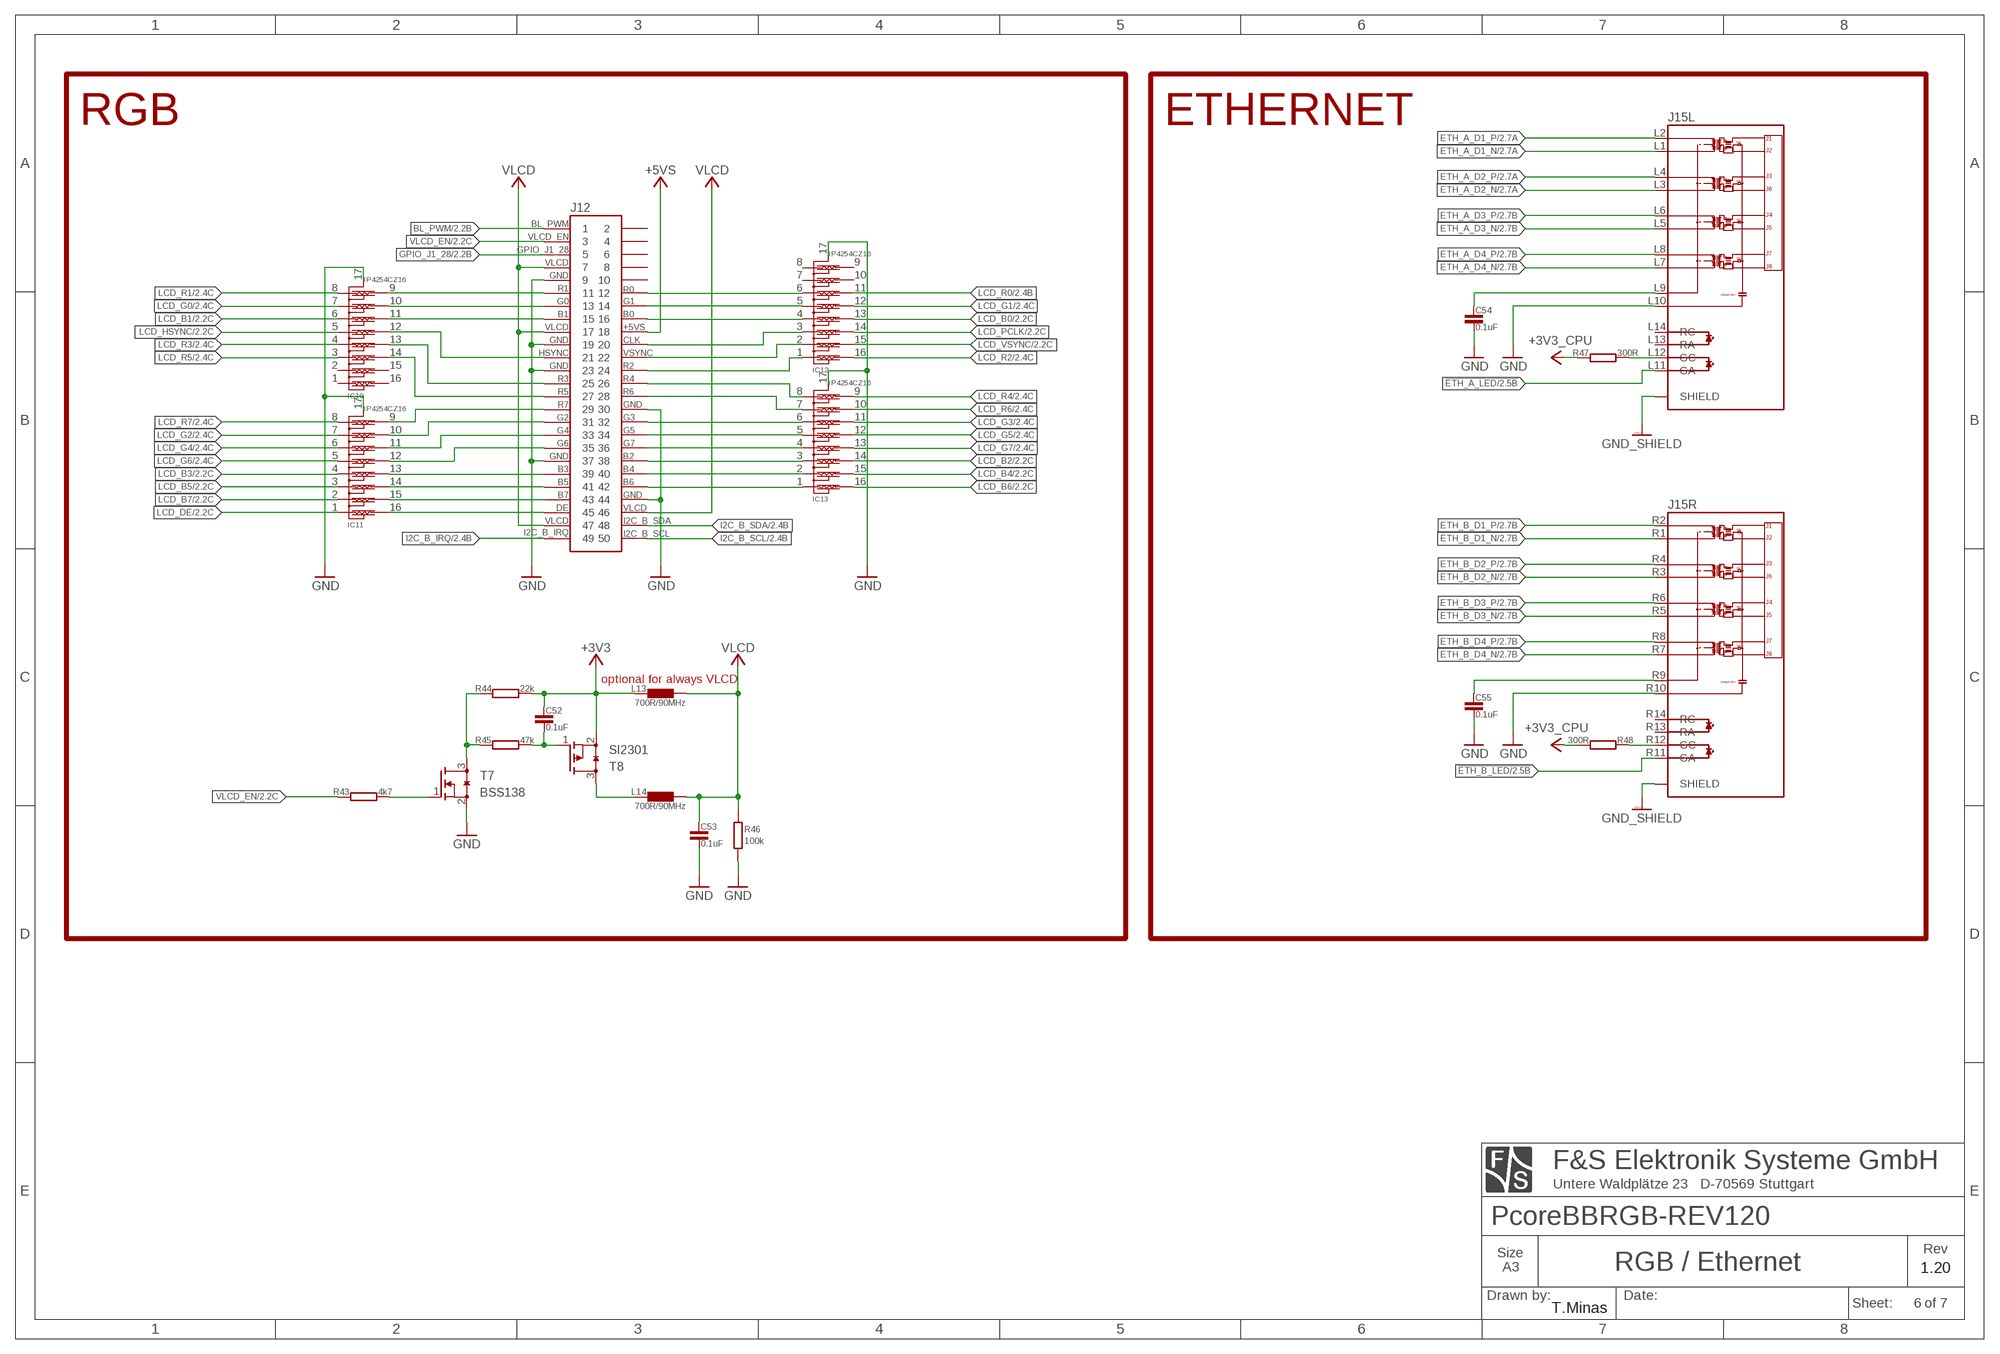
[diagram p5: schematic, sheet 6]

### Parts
C52  0.1uF  C0402-V  [0402@1]  (not fitted in variant FERT1B)
C53  0.1uF  C0402-V  [0402@1]  (not fitted in variant FERT1B)
C54  0.1uF  C0402-V  [0402@1]  (not fitted in variant FERT1B)
C55  0.1uF  C0402-V  [0402@1]  (not fitted in variant FERT1B)
IC10  IP4254CZ16  [SOT1168-1]  (not fitted in variant FERT1B)
IC11  IP4254CZ16  [SOT1168-1]  (not fitted in variant FERT1B)
IC12  IP4254CZ16  [SOT1168-1]  (not fitted in variant FERT1B)
IC13  IP4254CZ16  [SOT1168-1]  (not fitted in variant FERT1B)
J12  CON-DISPLAY-50-PCORE  [CON-DISPLAY-50-PCORE]  (not fitted in variant FERT1B)
J15  TRJG27440ADNL  [TRJG27440ADNL]
L13  700R/90MHz  L-EU-1206  [1206]  (not fitted in variant FERT1S)  (not fitted in variant FERT1B)
L14  700R/90MHz  L-EU-1206  [1206]  (not fitted in variant FERT1B)
R43  4k7  R0402  [0402]  (not fitted in variant FERT1B)
R44  22k  R0402  [0402]  (not fitted in variant FERT1B)
R45  47k  R0402  [0402]  (not fitted in variant FERT1B)
R46  100k  R0402-V  [0402@1]  (not fitted in variant FERT1B)
R47  300R  R0402  [0402]  (not fitted in variant FERT1B)
R48  300R  R0402  [0402]  (not fitted in variant FERT1B)
T7  BSS138  BSS138W  [SOT323(SC70)]  (not fitted in variant FERT1B)
T8  SI2301  SI2301DS  [SOT23]  (not fitted in variant FERT1B)

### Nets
!ETH_A_LED: J15.L11(L:GA) ; also sheet 2
+3V3 [+3V3]: C52.1 L13.1(IN) R44.2 T8.2(S) ; also sheet 3,4,5,7
+3V3_CPU [+3V3]: R47.1 R48.2 ; also sheet 2,3,7
+5VS: J12.18 ; also sheet 3,4,7
B0: IC12.4 J12.16
B1: IC10.11 J12.15
B2: IC13.3 J12.38
B3: IC11.13 J12.39
B4: IC13.2 J12.40
B5: IC11.14 J12.41
B6: IC13.1 J12.42
B7: IC11.15 J12.43
BL_PWM: J12.1 ; also sheet 2
CLK: IC12.3 J12.20
DE: IC11.16 J12.45
ETH_A_D1_N [ETHERNET]: J15.L1(L:TD1-) ; also sheet 2
ETH_A_D1_P [ETHERNET]: J15.L2(L:TD1+) ; also sheet 2
ETH_A_D2_N [ETHERNET]: J15.L3(L:TD2-) ; also sheet 2
ETH_A_D2_P [ETHERNET]: J15.L4(L:TD2+) ; also sheet 2
ETH_A_D3_N [ETHERNET]: J15.L5(L:TD3-) ; also sheet 2
ETH_A_D3_P [ETHERNET]: J15.L6(L:TD3+) ; also sheet 2
ETH_A_D4_N [ETHERNET]: J15.L7(L:TD4-) ; also sheet 2
ETH_A_D4_P [ETHERNET]: J15.L8(L:TD4+) ; also sheet 2
ETH_B_D1_N [ETHERNET]: J15.R1(R:TD1-) ; also sheet 2
ETH_B_D1_P [ETHERNET]: J15.R2(R:TD1+) ; also sheet 2
ETH_B_D2_N [ETHERNET]: J15.R3(R:TD2-) ; also sheet 2
ETH_B_D2_P [ETHERNET]: J15.R4(R:TD2+) ; also sheet 2
ETH_B_D3_N [ETHERNET]: J15.R5(R:TD3-) ; also sheet 2
ETH_B_D3_P [ETHERNET]: J15.R6(R:TD3+) ; also sheet 2
ETH_B_D4_N [ETHERNET]: J15.R7(R:TD4-) ; also sheet 2
ETH_B_D4_P [ETHERNET]: J15.R8(R:TD4+) ; also sheet 2
G0: IC10.10 J12.13
G1: IC12.5 J12.14
G2: IC11.10 J12.31
G3: IC13.6 J12.32
G4: IC11.11 J12.33
G5: IC13.5 J12.34
G6: IC11.12 J12.35
G7: IC13.4 J12.36
GND: C53.2 C54.2 C55.2 IC10.17 IC11.17 IC12.17 IC13.17 J12.9 J12.19 J12.23 J12.30 J12.37 J12.44 J15.L10(L:GND) J15.R10(R:GND) R46.1 T7.2(S) ; also sheet 1,2,3,4,5,7
GND_SHIELD: J15.SHIELD1(L:SHIELD) J15.SHIELD2(R:SHIELD) ; also sheet 1,3
GPIO_J1_28: J12.5 ; also sheet 2
HSYNC: IC10.12 J12.21
I2C_B_IRQ: J12.49 ; also sheet 2
I2C_B_SCL: J12.50 ; also sheet 2
I2C_B_SDA: J12.48 ; also sheet 2
LCD_B0: IC12.13 ; also sheet 2
LCD_B1: IC10.6 ; also sheet 2
LCD_B2: IC13.14 ; also sheet 2
LCD_B3: IC11.4 ; also sheet 2
LCD_B4: IC13.15 ; also sheet 2
LCD_B5: IC11.3 ; also sheet 2
LCD_B6: IC13.16 ; also sheet 2
LCD_B7: IC11.2 ; also sheet 2
LCD_DE: IC11.1 ; also sheet 2
LCD_G0: IC10.7 ; also sheet 2
LCD_G1: IC12.12 ; also sheet 2
LCD_G2: IC11.7 ; also sheet 2
LCD_G3: IC13.11 ; also sheet 2
LCD_G4: IC11.6 ; also sheet 2
LCD_G5: IC13.12 ; also sheet 2
LCD_G6: IC11.5 ; also sheet 2
LCD_G7: IC13.13 ; also sheet 2
LCD_HSYNC: IC10.5 ; also sheet 2
LCD_PCLK: IC12.14 ; also sheet 2
LCD_R0: IC12.11 ; also sheet 2
LCD_R1: IC10.8 ; also sheet 2
LCD_R2: IC12.16 ; also sheet 2
LCD_R3: IC10.4 ; also sheet 2
LCD_R4: IC13.9 ; also sheet 2
LCD_R5: IC10.3 ; also sheet 2
LCD_R6: IC13.10 ; also sheet 2
LCD_R7: IC11.8 ; also sheet 2
LCD_VSYNC: IC12.15 ; also sheet 2
N$3: C55.1 J15.R9(R:VCC)
N$6: J15.L12(L:GC) R47.2
N$7: J15.R12(R:GC) R48.1
N$41: C54.1 J15.L9(L:VCC)
N$120: R43.2 T7.1(G)
N$121: R44.1 R45.1 T7.3(D)
N$124: C52.2 R45.2 T8.1(G)
N$126: L14.1(IN) T8.3(D)
R0: IC12.6 J12.12
R1: IC10.9 J12.11
R2: IC12.1 J12.24
R3: IC10.13 J12.25
R4: IC13.8 J12.26
R5: IC10.14 J12.27
R6: IC13.7 J12.28
R7: IC11.9 J12.29
VLCD: C53.1 J12.7 J12.17 J12.46 J12.47 L13.2(OUT) L14.2(OUT) R46.2
VLCD_EN: J12.3 R43.1 ; also sheet 2
VSYNC: IC12.2 J12.22
Unconnected: IC10.1 IC10.2 IC10.15 IC10.16 IC12.7 IC12.8 IC12.9 IC12.10 J12.2 J12.4 J12.6 J12.8 J12.10 J15.L13(L:RA) J15.L14(L:RC) J15.R11(R:GA) J15.R13(R:RA) J15.R14(R:RC)

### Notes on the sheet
- RGB | ETHERNET
- optional for always VLCD
- 1.20
- T.Minas

## Sheet 7 of 7: DC/DC
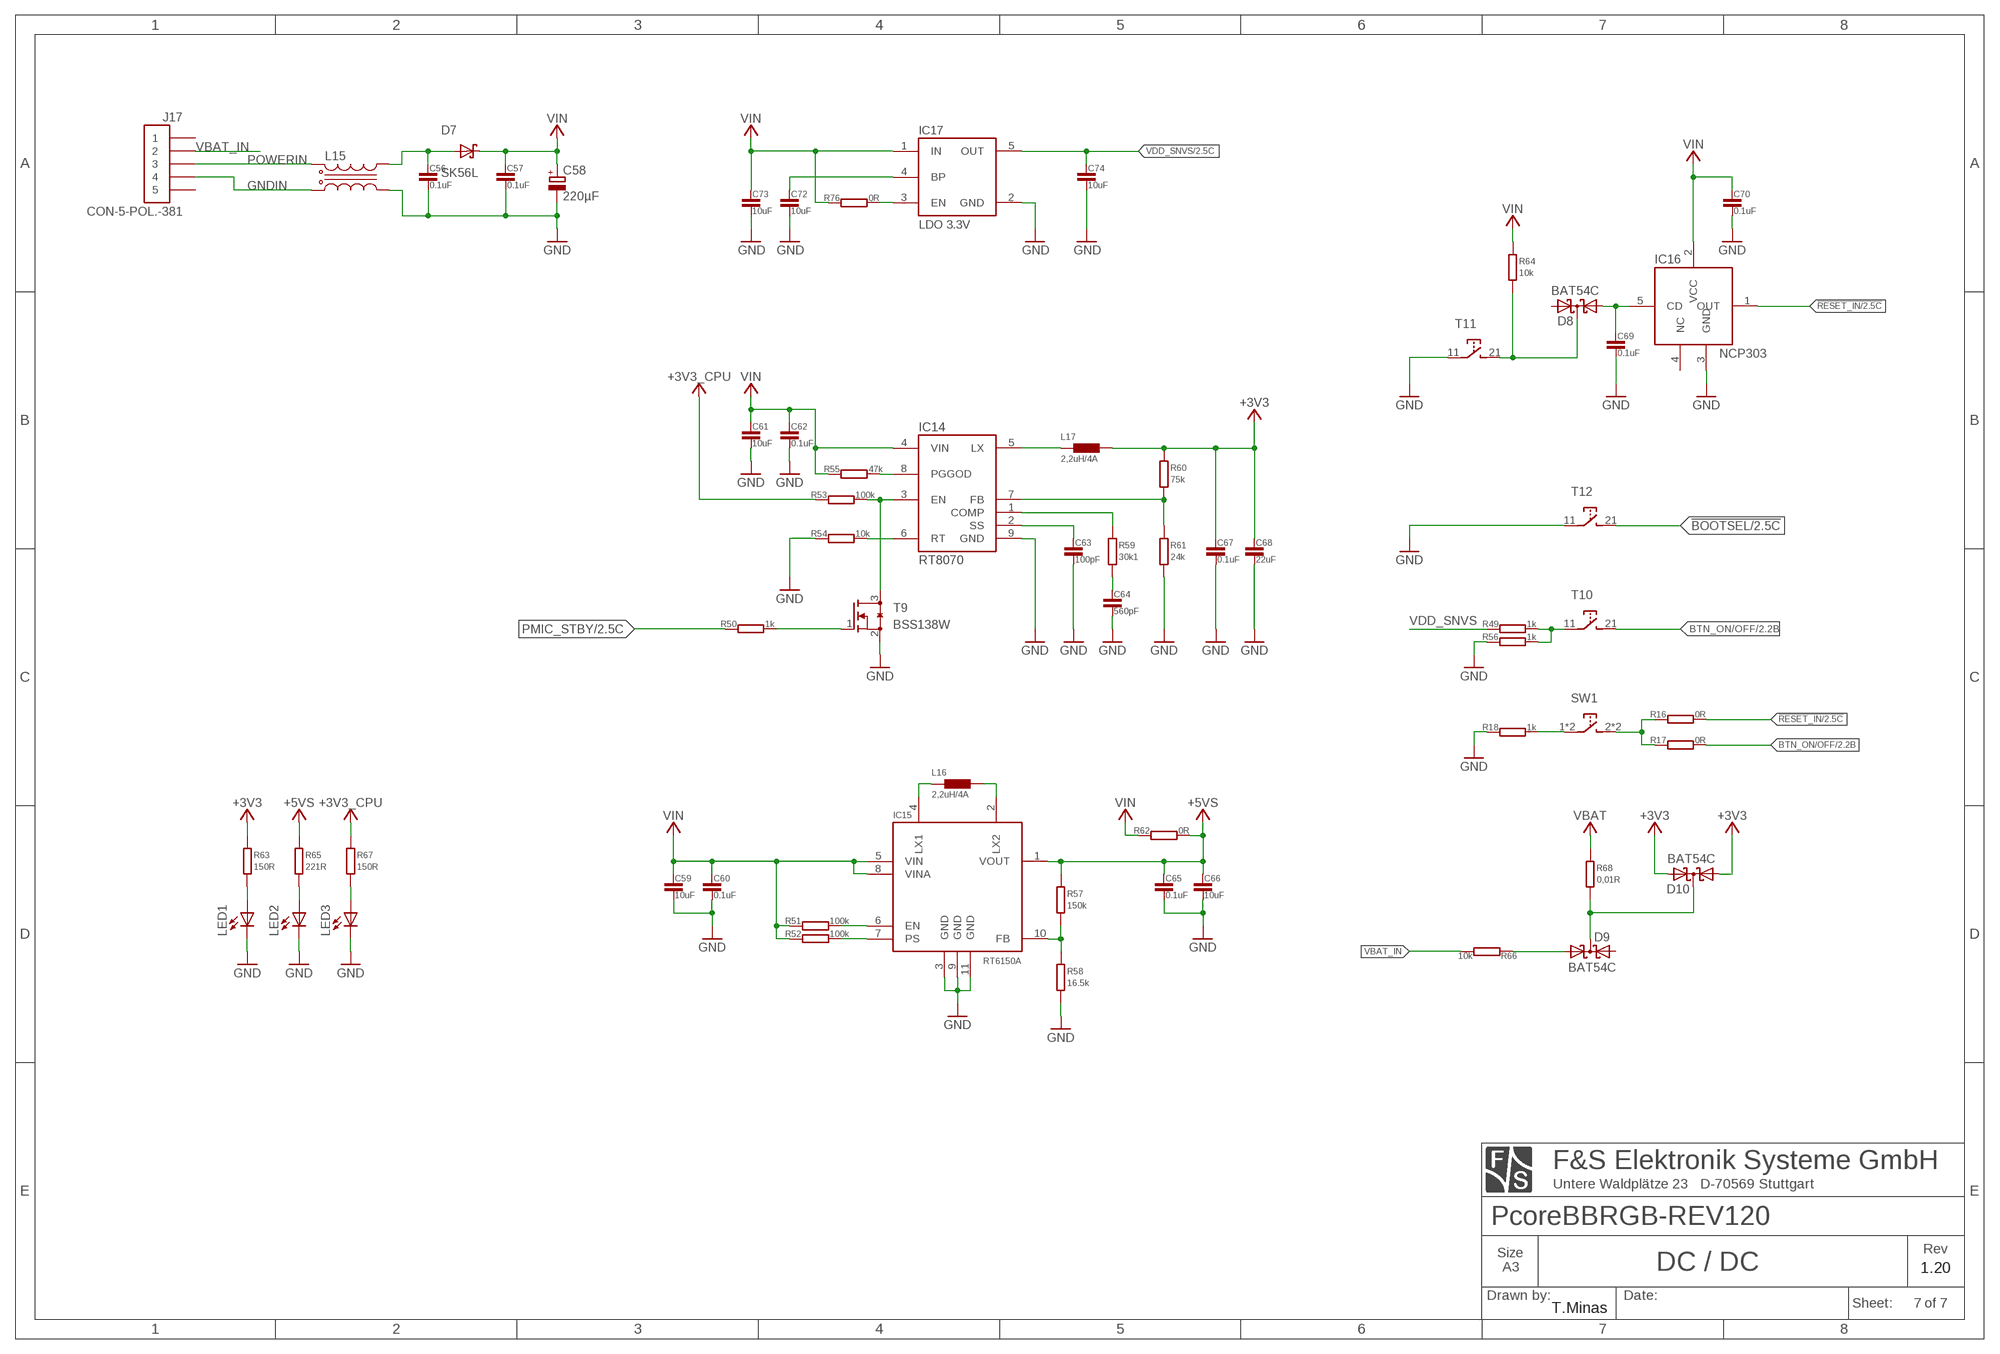
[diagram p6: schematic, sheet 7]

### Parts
C56  0.1uF  C0402-V  [0402@1]  (not fitted in variant FERT1B)
C57  0.1uF  C0402-V  [0402@1]  (not fitted in variant FERT1B)
C58  220µF  CPOL-EUSMCD  [SMC_D]  (not fitted in variant FERT1B)
C59  10uF  C0603-V  [0603]  (not fitted in variant FERT1B)
C60  0.1uF  C0402-V  [0402@1]  (not fitted in variant FERT1B)
C61  10uF  C0603-V  [0603]  (not fitted in variant FERT1B)
C62  0.1uF  C0402-V  [0402@1]  (not fitted in variant FERT1B)
C63  100pF  C0402-V  [0402@1]  (not fitted in variant FERT1B)
C64  560pF  C0402-V  [0402@1]  (not fitted in variant FERT1B)
C65  0.1uF  C0402-V  [0402@1]  (not fitted in variant FERT1B)
C66  10uF  C0603-V  [0603]  (not fitted in variant FERT1B)
C67  0.1uF  C0402-V  [0402@1]  (not fitted in variant FERT1B)
C68  22uF  C0805-V  [0805]  (not fitted in variant FERT1B)
C69  0.1uF  C0402-V  [0402@1]  (not fitted in variant FERT1B)
C70  0.1uF  C0402-V  [0402@1]  (not fitted in variant FERT1B)
C72  10uF  C0402-V  [0402@1]  (not fitted in variant FERT1B)
C73  10uF  C0402-V  [0402@1]  (not fitted in variant FERT1B)
C74  10uF  C0402-V  [0402@1]
D7  SK56L  D-SK52L  [D-DO214AB(SMC)]  (not fitted in variant FERT1B)
D8  BAT54C  [SOT23]  (not fitted in variant FERT1B)
D9  BAT54C  [SOT23]  (not fitted in variant FERT1B)
D10  BAT54C  [SOT23]  (not fitted in variant FERT1B)
IC14  RT8070  RT8070ZQW  [WDFN-8L]  (not fitted in variant FERT1B)
IC15  RT6150A  [WDFN-10L3X3]  (not fitted in variant FERT1B)
IC16  NCP303  NCP303LSN30T1G  [SOT23-5]  (not fitted in variant FERT1B)
IC17  LDO 3.3V  AP7365  [SOT23-5]  (not fitted in variant FERT1B)
J17  CON-5-POL.-381  [CON-5-POL.]
L15  L-WE-SL5  [L-WE-SL5]  (not fitted in variant FERT1B)
L16  2,2uH/4A  L-VLC5045  [VLC5045]  (not fitted in variant FERT1B)
L17  2,2uH/4A  L-VLC5045  [VLC5045]  (not fitted in variant FERT1B)
LED1  LED0603  [LED0603]  (not fitted in variant FERT1B)
LED2  LED0603  [LED0603]  (not fitted in variant FERT1B)
LED3  LED0603  [LED0603]  (not fitted in variant FERT1B)
R16  0R  R0402  [0402]
R17  0R  R0402  [0402]
R18  1k  R0402  [0402]
R49  1k  R0402  [0402]  (not fitted in variant FERT1S)  (not fitted in variant FERT1B)
R50  1k  R0402  [0402]  (not fitted in variant FERT1B)
R51  100k  R0402  [0402]  (not fitted in variant FERT1B)
R52  100k  R0402  [0402]  (not fitted in variant FERT1B)
R53  100k  R0402  [0402]  (not fitted in variant FERT1B)
R54  10k  R0402  [0402]  (not fitted in variant FERT1B)
R55  47k  R0402  [0402]  (not fitted in variant FERT1B)
R56  1k  R0402  [0402]  (not fitted in variant FERT1B)
R57  150k  R0402-V  [0402@1]  (not fitted in variant FERT1B)
R58  16.5k  R0402-V  [0402@1]  (not fitted in variant FERT1B)
R59  30k1  R0402-V  [0402@1]  (not fitted in variant FERT1B)
R60  75k  R0402-V  [0402@1]  (not fitted in variant FERT1B)
R61  24k  R0402-V  [0402@1]  (not fitted in variant FERT1B)
R62  0R  R0805-H  [0805]  (not fitted in variant FERT1B)  (not fitted in variant FERT1S)
R63  150R  R0402-V  [0402@1]  (not fitted in variant FERT1B)
R64  10k  R0402-V  [0402@1]  (not fitted in variant FERT1B)
R65  221R  R0402-V  [0402@1]  (not fitted in variant FERT1B)
R66  10k  R0402  [0402]  (not fitted in variant FERT1B)
R67  150R  R0402-V  [0402@1]  (not fitted in variant FERT1B)
R68  0,01R  R0805-V  [0805]  (not fitted in variant FERT1B)
R76  0R  R0402  [0402]  (not fitted in variant FERT1B)
SW1  TASTER-WE-SEITE  [TASTER-WE-436351045816]
T9  BSS138W  [SOT323(SC70)]  (not fitted in variant FERT1B)
T10  TASTER_SMD  [TASTER_SMD]  (not fitted in variant FERT1B)
T11  TASTER_SMD  [TASTER_SMD]  (not fitted in variant FERT1B)
T12  TASTER_SMD  [TASTER_SMD]  (not fitted in variant FERT1B)

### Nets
!BOOTSEL: T12.21(OUT) ; also sheet 2
!RESET_BTN: D8.3(CC) R64.1 T11.21(OUT)
!RESET_IN: IC16.1(OUT) R16.2 ; also sheet 2,3
+3V3 [+3V3]: C67.1 C68.1 D10.1(A1) D10.2(A2) L17.2(OUT) R60.2 R63.2 ; also sheet 3,4,5,6
+3V3_CPU [+3V3]: R53.1 R67.2 ; also sheet 2,3,6
+5VS: C65.1 C66.1 IC15.1(VOUT) R57.2 R62.2 R65.2 ; also sheet 3,4,6
BTN_ON/OFF: R17.2 T10.21(OUT) ; also sheet 2
GND: C56.2 C57.2 C58.- C59.2 C60.2 C61.2 C62.2 C63.2 C64.2 C65.2 C66.2 C67.2 C68.2 C69.2 C70.2 C72.2 C73.2 C74.2 IC14.9(GND) IC15.3(GND) IC15.9(GND) IC15.11(GND) IC16.3(GND) IC17.2(GND) L15.3 LED1.C LED2.C LED3.C R18.1 R54.1 R56.1 R58.1 R61.1 T9.2(S) T11.11(IN) T12.11(IN) ; also sheet 1,2,3,4,5,6
GNDIN: J17.4 L15.4
N$5: C69.1 D8.1(A1) IC16.5(CD)
N$22: R50.2 T9.1(G)
N$36: C56.1 D7.2(A) L15.2
N$37: R16.1 R17.1 SW1.2(OUT) SW1.4(OUT)
N$44: LED1.A R63.1
N$47 [+3V3]: IC17.3(EN) R76.2
N$48: C72.1 IC17.4(BP)
N$49: R49.2 R56.2 T10.11(IN)
N$53: IC14.6(RT) R54.2
N$58: R18.2 SW1.1(IN) SW1.3(IN)
N$63: LED2.A R65.1
N$64: IC15.4(LX1) L16.1(IN)
N$65: IC15.2(LX2) L16.2(OUT)
N$66: LED3.A R67.1
N$67: IC15.6(EN) R51.2
N$68: IC15.7(PS) R52.2
N$72: IC15.10(FB) R57.1 R58.2
N$75: C64.1 R59.1
N$76: C63.1 IC14.2(SS)
N$78: IC14.3(EN) R53.2 T9.3(D)
N$79: IC14.8(PGGOD) R55.2
N$84: IC14.1(COMP) R59.2
N$85: IC14.7(FB) R60.1 R61.2
N$90: IC14.5(LX) L17.1(IN)
N$141: D9.1(A1) R66.1
N$142: D9.3(CC) D10.3(CC) R68.1
PMIC_STBY: R50.1 ; also sheet 2
POWERIN: J17.3 L15.1
VBAT: R68.2 ; also sheet 2
VBAT_IN: J17.2 R66.2
VDD_SNVS: C74.1 IC17.5(OUT) R49.1 ; also sheet 2
VIN: C57.1 C58.+ C59.1 C60.1 C61.1 C62.1 C70.1 C73.1 D7.1(C) IC14.4(VIN) IC15.5(VIN) IC15.8(VINA) IC16.2(VCC) IC17.1(IN) R51.1 R52.1 R55.1 R62.1 R64.2 R76.1 ; also sheet 2,5
Unconnected: D8.2(A2) D9.2(A2) IC16.4(NC) J17.1 J17.5

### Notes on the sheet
- 1.20
- T.Minas

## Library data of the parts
A-REF1-A-REF6 = F&SElektronikSysteme:A-REF
BQ1 = F&SElektronikSysteme:Q-FA-238
C1 C2 = F&SElektronikSysteme:C1206-H
C3 C8-C15 C17 C20-C26 C33-C43 C46-C57 C60 C62-C65 C67 C69-C74 C76-C80 = F&SElektronikSysteme:C0402-V
C5 C6 C27-C32 = F&SElektronikSysteme:C0402
C18 C19 C58 C75 = resistor:CPOL-EU: POLARIZED CAPACITOR, European symbol
C44 C45 = F&SElektronikSysteme:C0603-H
C59 C61 C66 = F&SElektronikSysteme:C0603-V
C68 = F&SElektronikSysteme:C0805-V
D1 D3 D8-D10 = F&SElektronikSysteme:BAT54C: Schottky Diodes Source: Fairchild .. BAT54.pdf
D4-D6 = F&SElektronikSysteme:PGB1SOT23
D7 = F&SElektronikSysteme:D-SK52L
D11 = F&SElektronikSysteme:ESD-PROTECTION-DIODE(4CHANNEL)
D12 = F&SElektronikSysteme:RB521S30
F1 = F&SElektronikSysteme:F-EU-0805
H1-H4 = F&SElektronikSysteme:HOLE-3.2X6
IC2 = F&SElektronikSysteme:USB2422
IC4 = F&SElektronikSysteme:MIC2026
IC5 IC6 = F&SElektronikSysteme:SP3232ECY
IC7 = F&SElektronikSysteme:TJA1051T/3
IC8 = F&SElektronikSysteme:ADP171
IC9 IC17 = F&SElektronikSysteme:AP7365
IC10-IC13 = F&SElektronikSysteme:IP4254CZ16
IC14 = F&SElektronikSysteme:RT8070ZQW
IC15 = F&SElektronikSysteme:RT6150A
IC16 = F&SElektronikSysteme:NCP303LSN30T1G
IC18 = F&SElektronikSysteme:TPS2051BDBV
J1 = F&SElektronikSysteme:CON-MINI-USB-SCHIELD: MINI USB-B Conector Source: www.cypressindustries.com; OC_FARNELL: unknown; OC_NEWARK: unknown
J2 = F&SElektronikSysteme:CON-10-POL.-SMD-127
J4 = F&SElektronikSysteme:CON-USB-DOUBLE
J5-J8 = F&SElektronikSysteme:CON-10-POL.-STIFTWANNE-B
J9 = F&SElektronikSysteme:CON-50-POL.
J10 = F&SElektronikSysteme:CON-MICRO-SD-PUSHPULL
J11 = F&SElektronikSysteme:CON-AUDIO-HP-MIC
J12 = F&SElektronikSysteme:CON-DISPLAY-50-PCORE
J15 = F&SElektronikSysteme:TRJG27440ADNL
J16 = F&SElektronikSysteme:CON-HIROSE-DF13A-6P
J17 = F&SElektronikSysteme:CON-5-POL.-381
L1 L6 L7 = Wuerth_Elektronik_eiSos_V6:WE-CNSW_HF: SMD Common Mode Noise Suppressor WE-CNSW HF - High common mode suppression at high frequency - Small influence for high speed signals through winding symmetry - Suitable for high data rates -- USB 3.0 -- Firewire / IEEE 1394 -- HDMI -- High Speed Data Lines -- LVDS -- Common mode data line filter
L4 L5 L10-L12 = Wuerth_Elektronik_eiSos_V6:WE-CBF_HF: SMD EMI Suppression Ferrite Beads WE-CBF HF
L8 L9 L18 = F&SElektronikSysteme:L-EU-0603
L13 L14 L20 = F&SElektronikSysteme:L-EU-1206
L15 = F&SElektronikSysteme:L-WE-SL5
L16 L17 = F&SElektronikSysteme:L-VLC5045
L19 = WE:WE-CNSW: SMD Common Mode Noise Suppressor WE-CNSW - High common mode suppression at high frequency - Small influence for high speed signals through winding symmetry -- USB 2.0 -- Firewire / IEEE 1394 -- Power supply systems -- High Speed Data Lines -- Common mode data line filter
LED1-LED3 = F&SElektronikSysteme:LED0603
PCORE_ = F&SElektronikSysteme:PICOCORE
R1 R10 R62 = F&SElektronikSysteme:R0805-H
R2-R7 R12-R18 R20-R26 R36 R43-R45 R47-R56 R66 R70-R73 R76 R81 R82 = F&SElektronikSysteme:R0402
R8 R9 R11 R27-R35 R37-R42 R46 R57-R61 R63-R65 R67 R74 R75 R77-R80 = F&SElektronikSysteme:R0402-V
R68 = F&SElektronikSysteme:R0805-V
SW1 = F&SElektronikSysteme:TASTER-WE-SEITE
T2 T4-T7 T9 T13 = F&SElektronikSysteme:BSS138W
T3 T8 = F&SElektronikSysteme:SI2301DS
T10-T12 = F&SElektronikSysteme:TASTER_SMD
T14 = F&SElektronikSysteme2:SI2301DS
T15 = F&SElektronikSysteme2:BSS138W
TP1 = F&SElektronikSysteme:TEST2

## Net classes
0 default: width 0.1 mm, drill 0.2 mm, clearance 0.1 mm
1 USB: width 0.161 mm, drill 0.2 mm, clearance 0.5 mm to class 0, clearance 0.1 mm
2 ETHERNET: width 0.127 mm, drill 0.2 mm, clearance 0.5 mm to class 0, clearance 0.5 mm to class 1, clearance 0.1 mm
3 +3V3: width 0.1 mm, drill 0.2 mm, clearance 0.1 mm to class 0, clearance 0.5 mm to class 1, clearance 0.5 mm to class 2, clearance 0.1 mm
